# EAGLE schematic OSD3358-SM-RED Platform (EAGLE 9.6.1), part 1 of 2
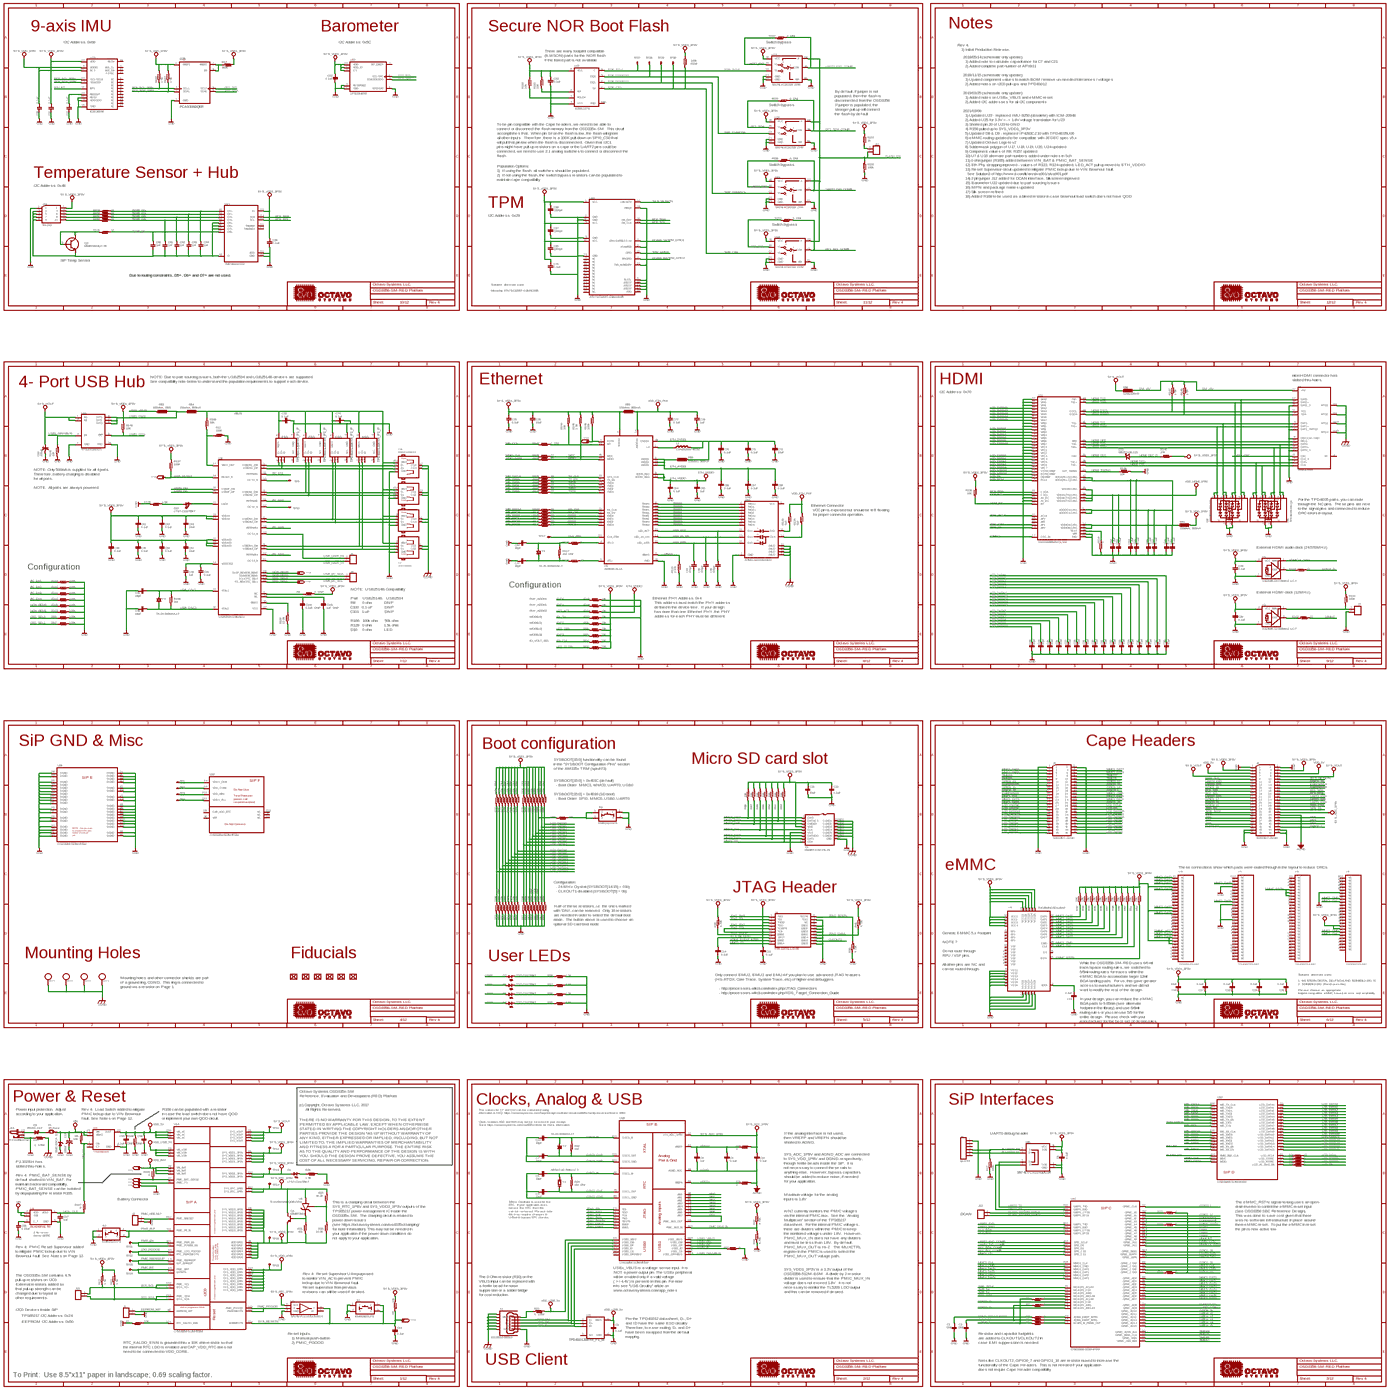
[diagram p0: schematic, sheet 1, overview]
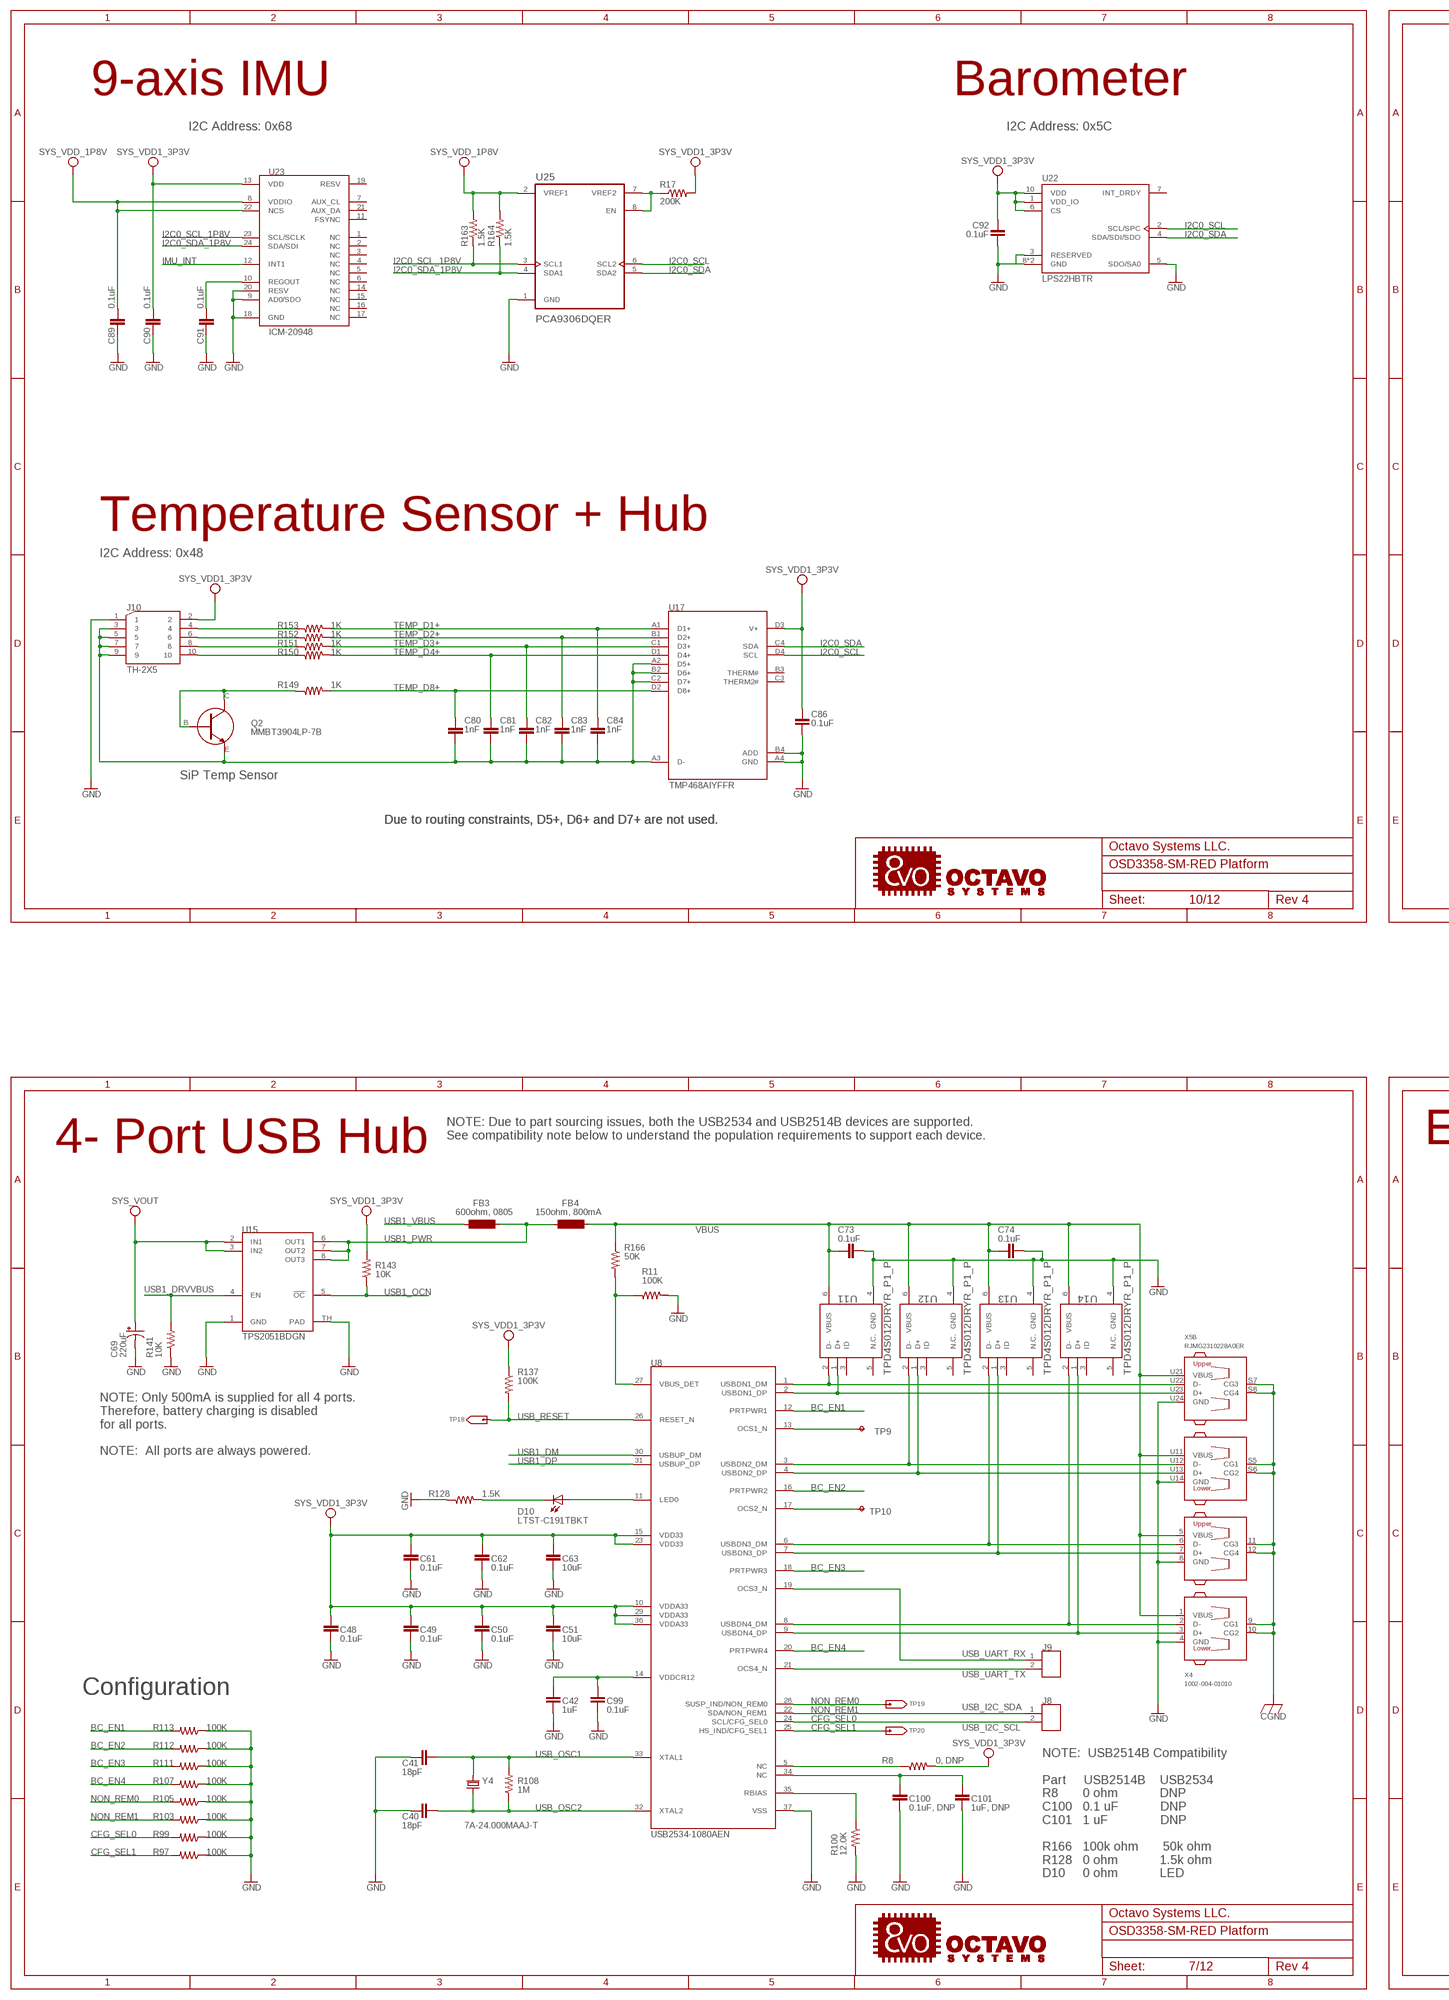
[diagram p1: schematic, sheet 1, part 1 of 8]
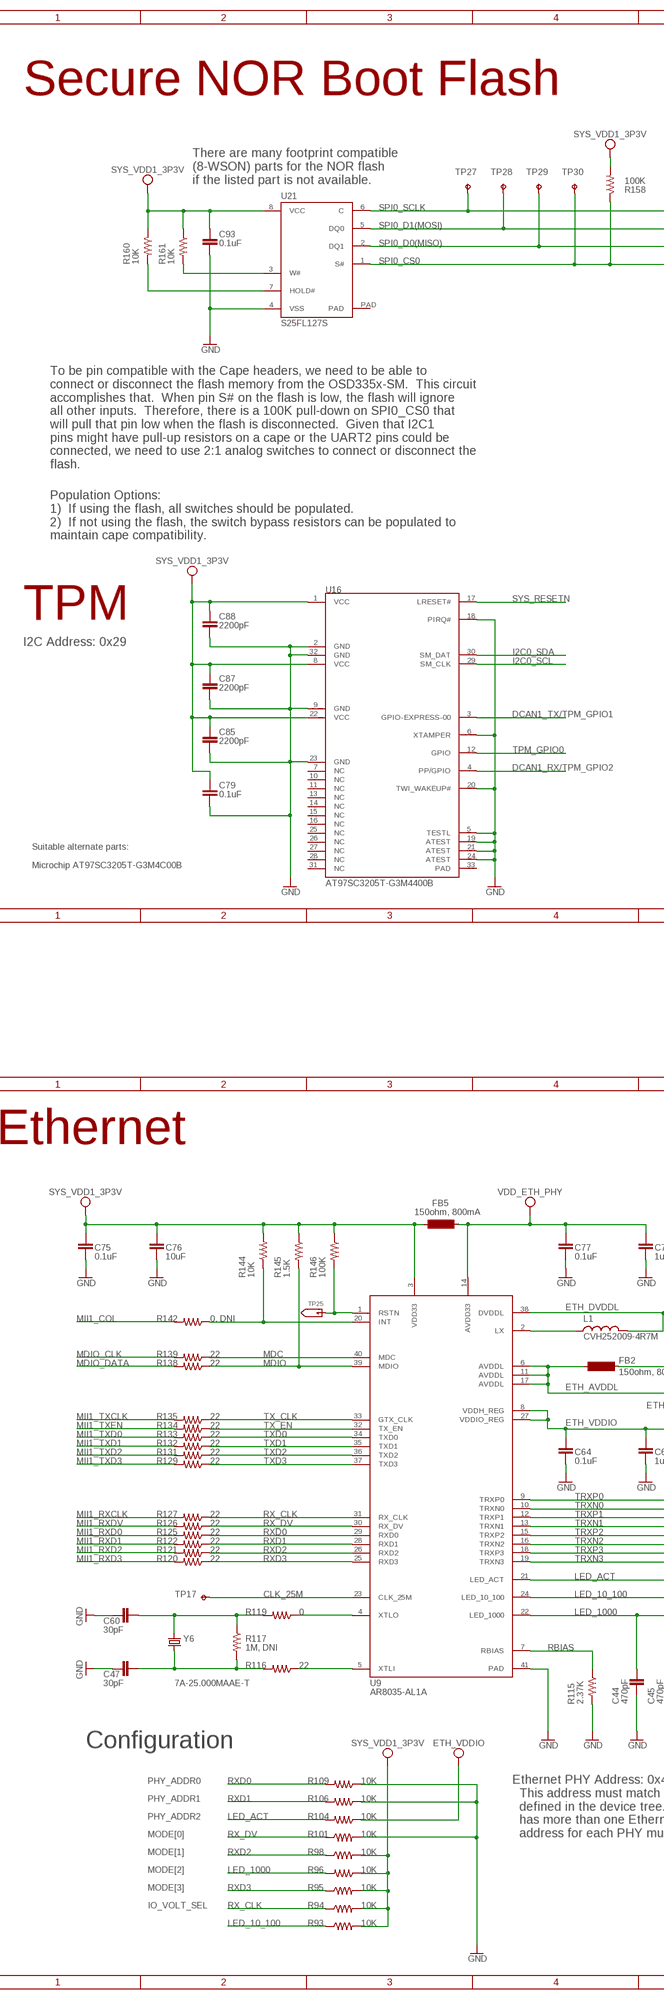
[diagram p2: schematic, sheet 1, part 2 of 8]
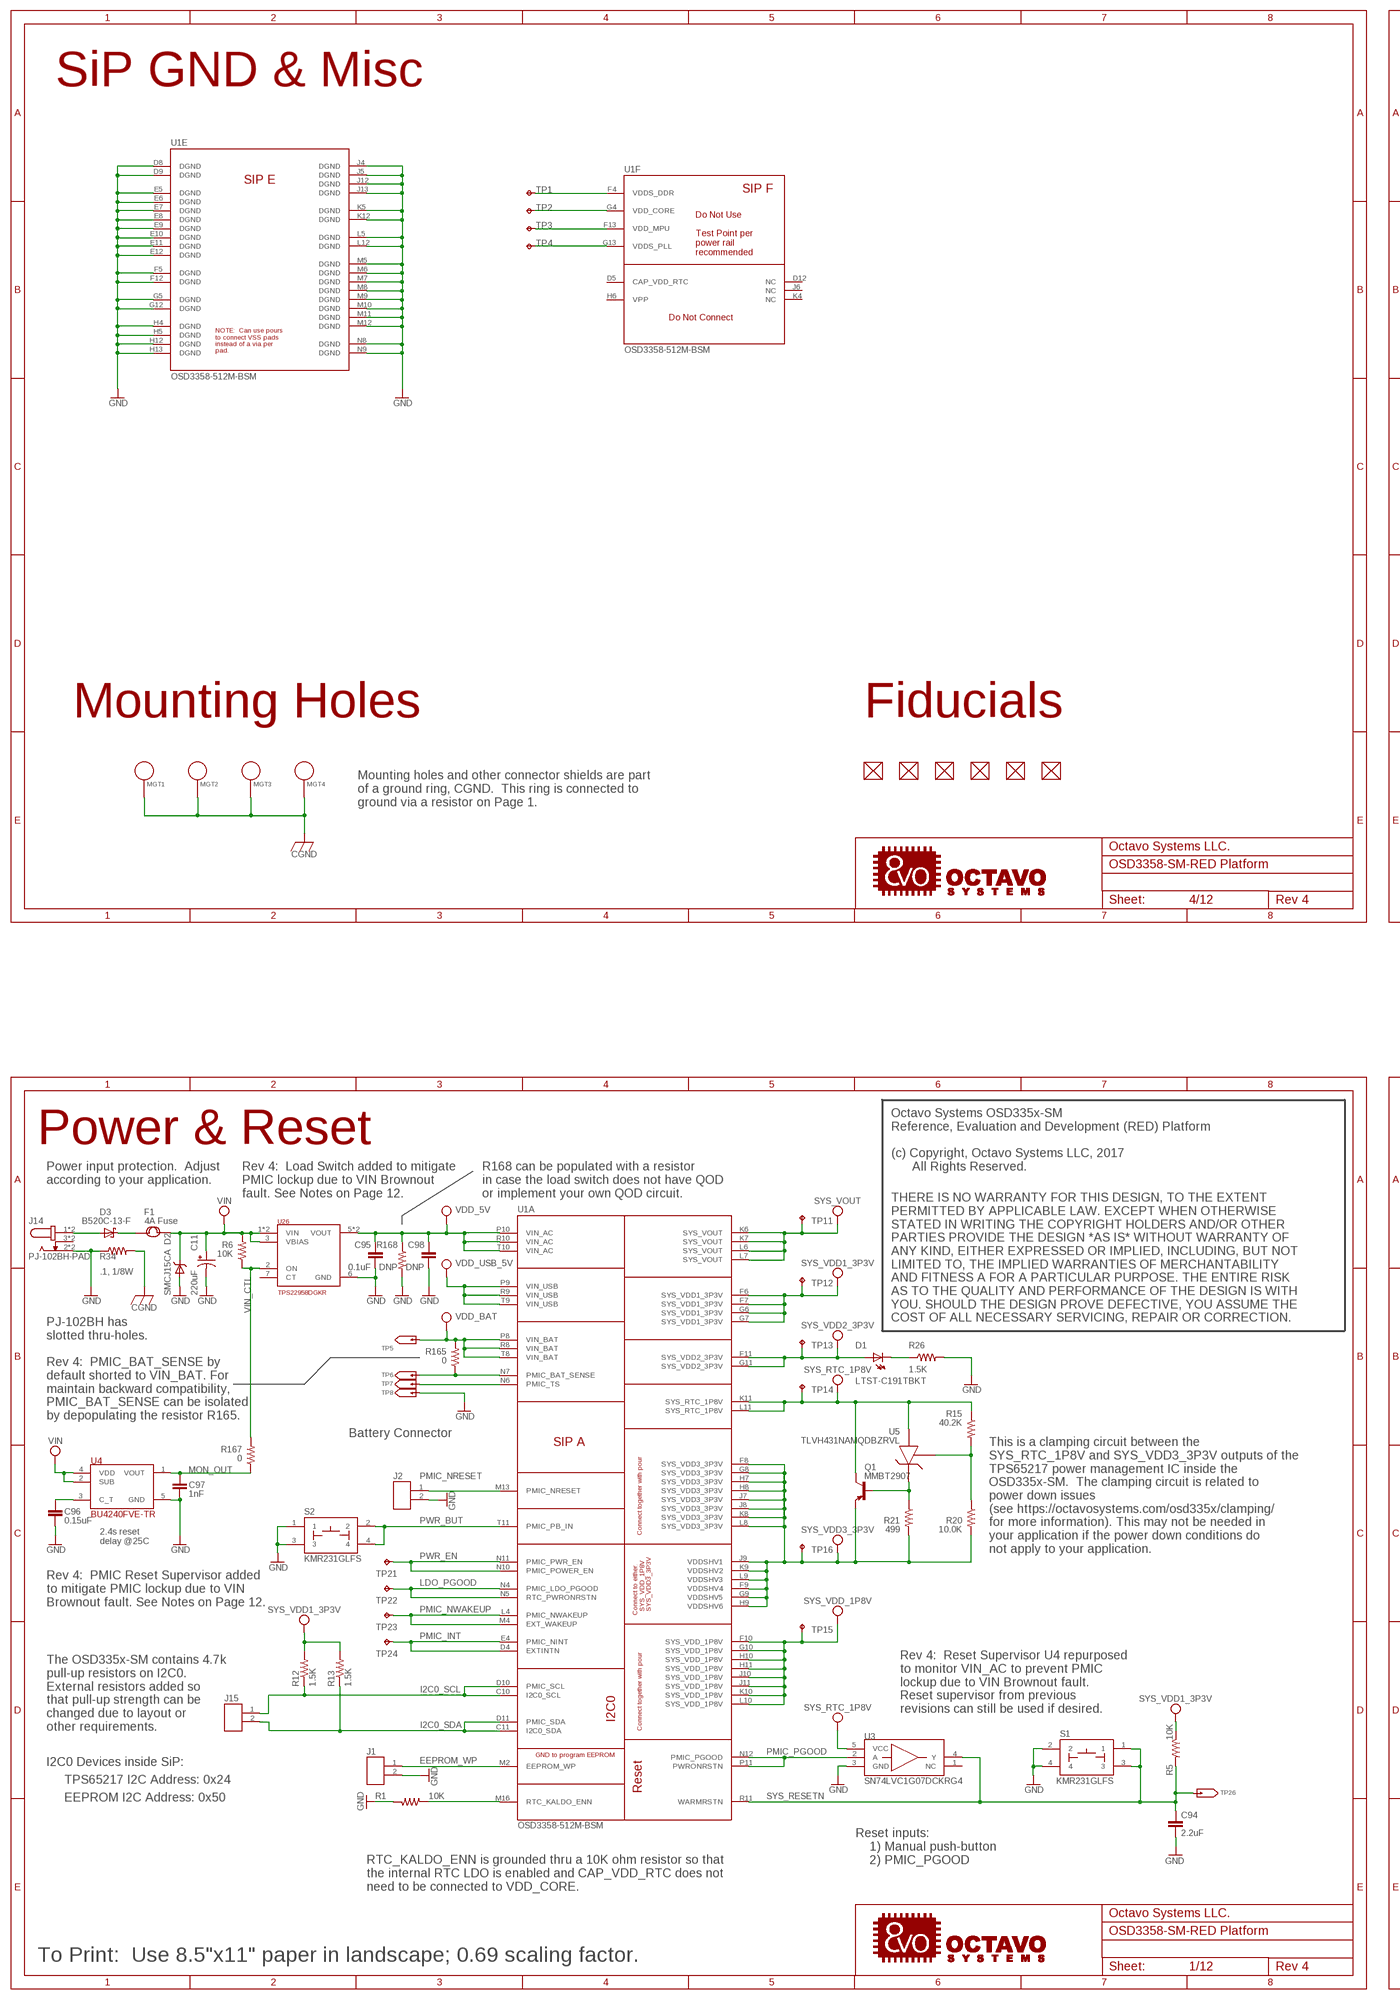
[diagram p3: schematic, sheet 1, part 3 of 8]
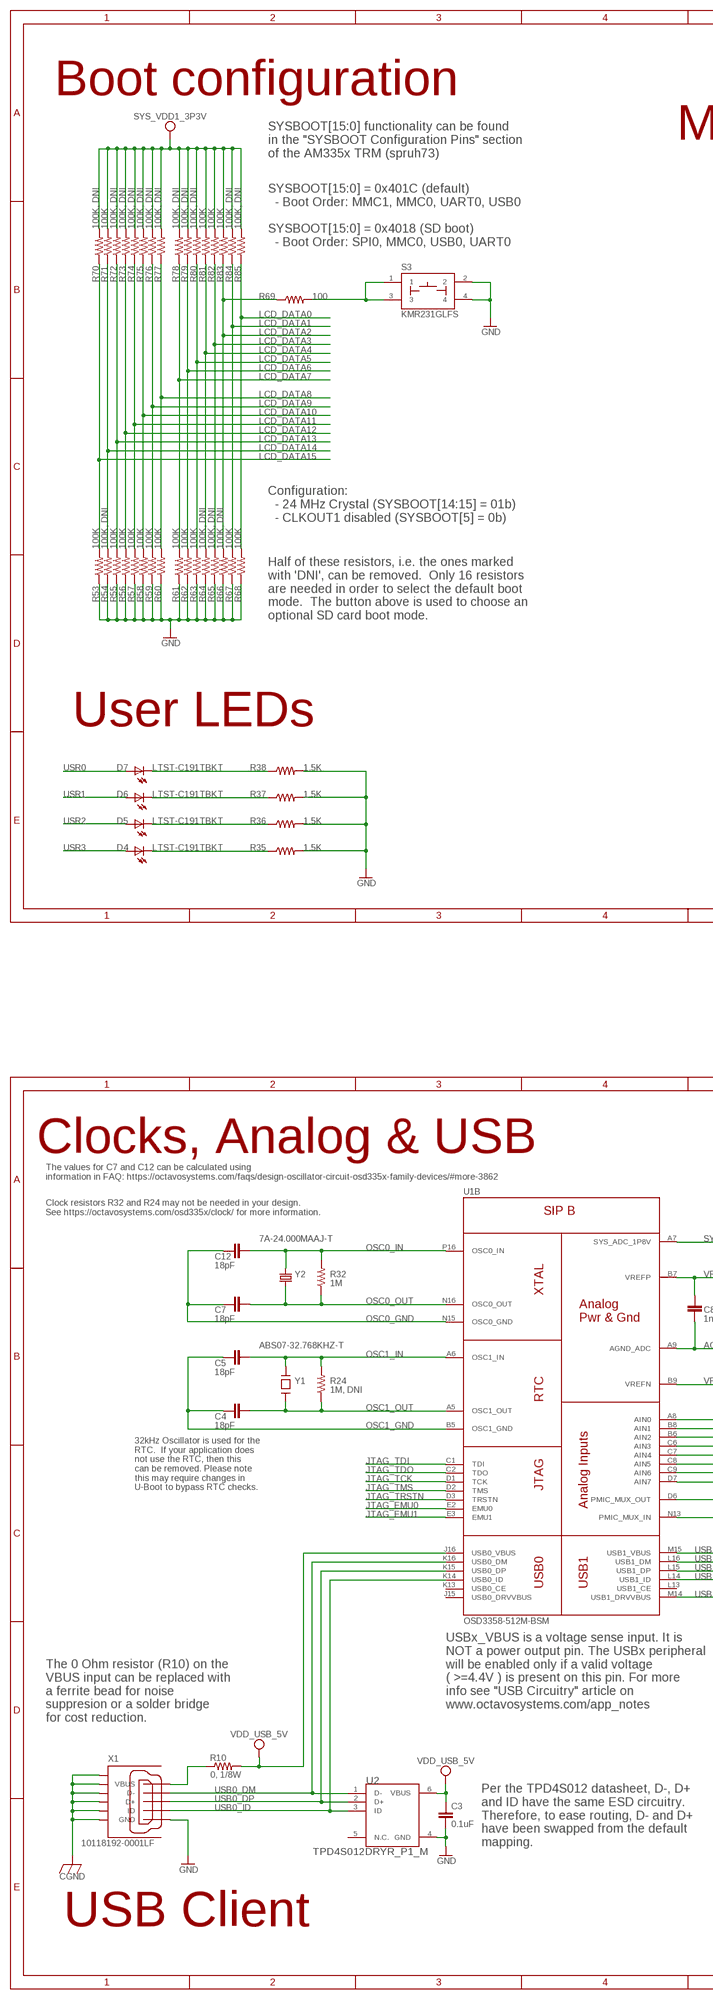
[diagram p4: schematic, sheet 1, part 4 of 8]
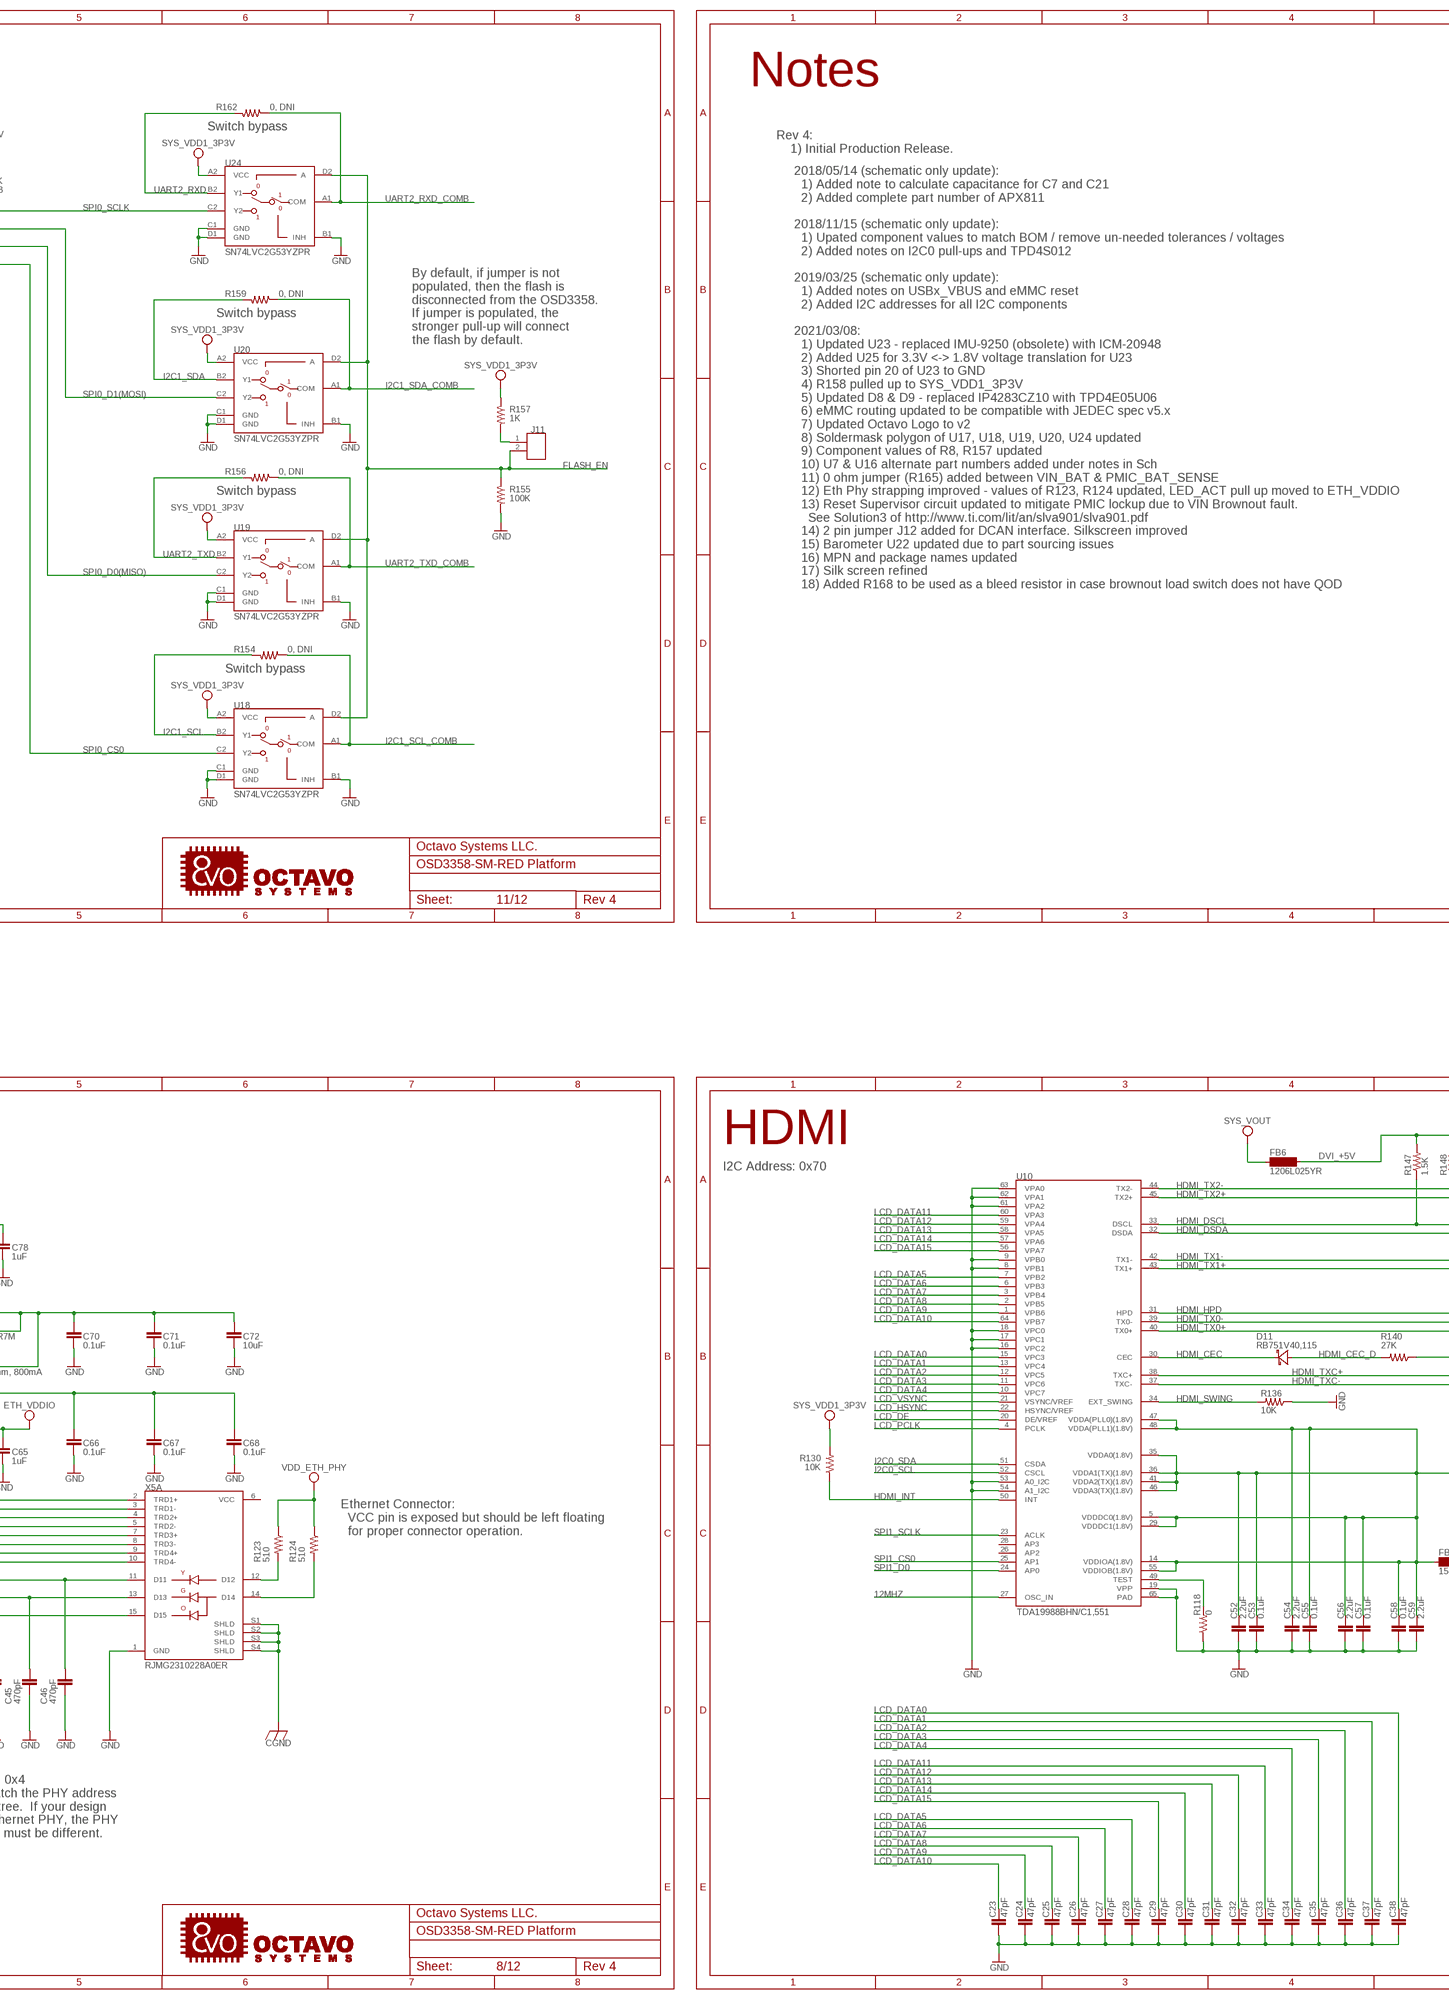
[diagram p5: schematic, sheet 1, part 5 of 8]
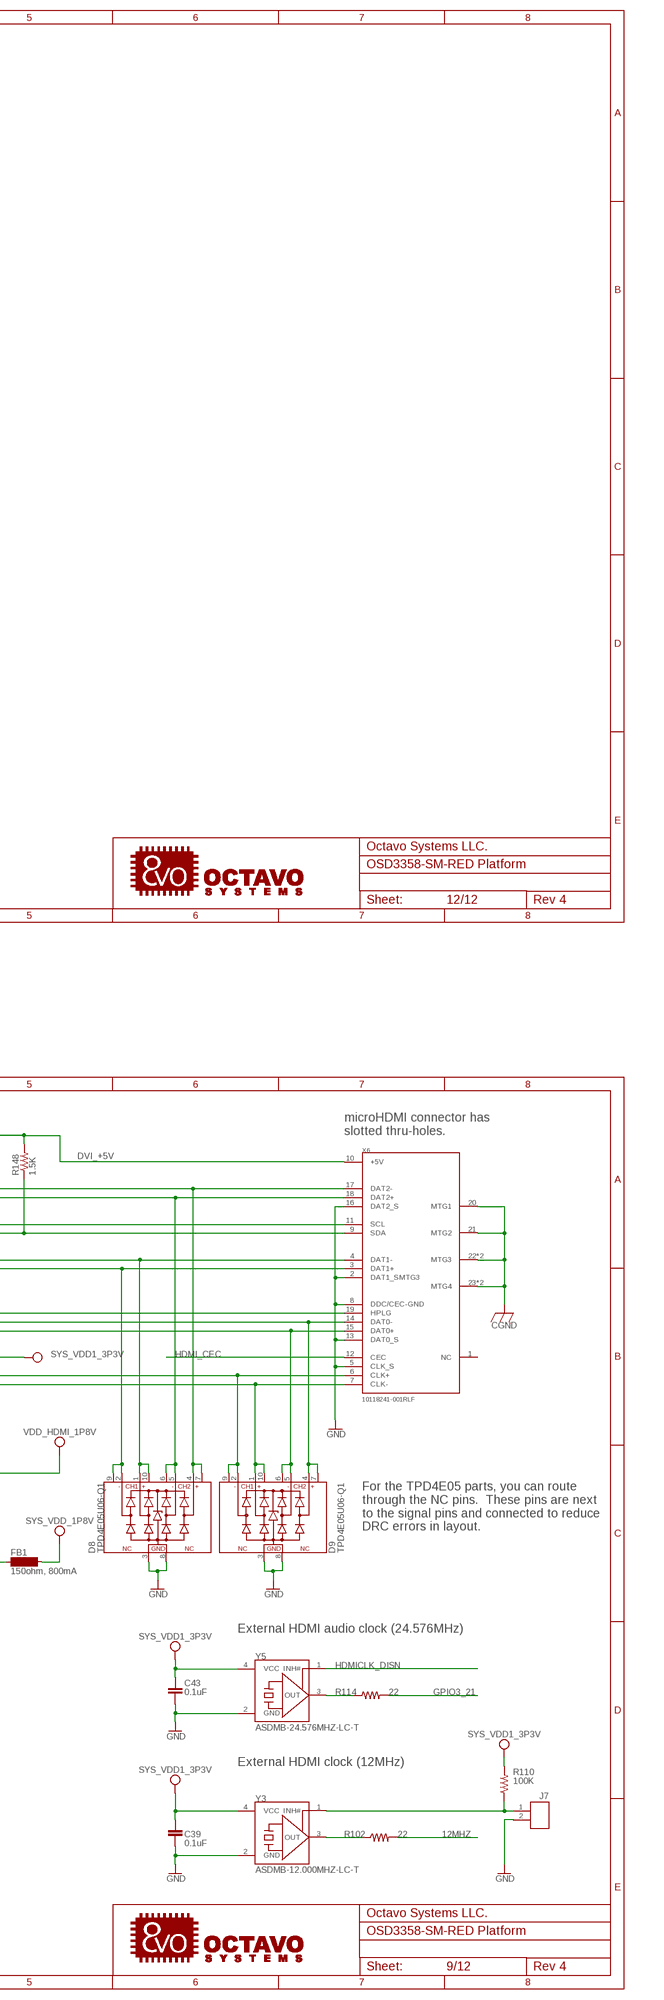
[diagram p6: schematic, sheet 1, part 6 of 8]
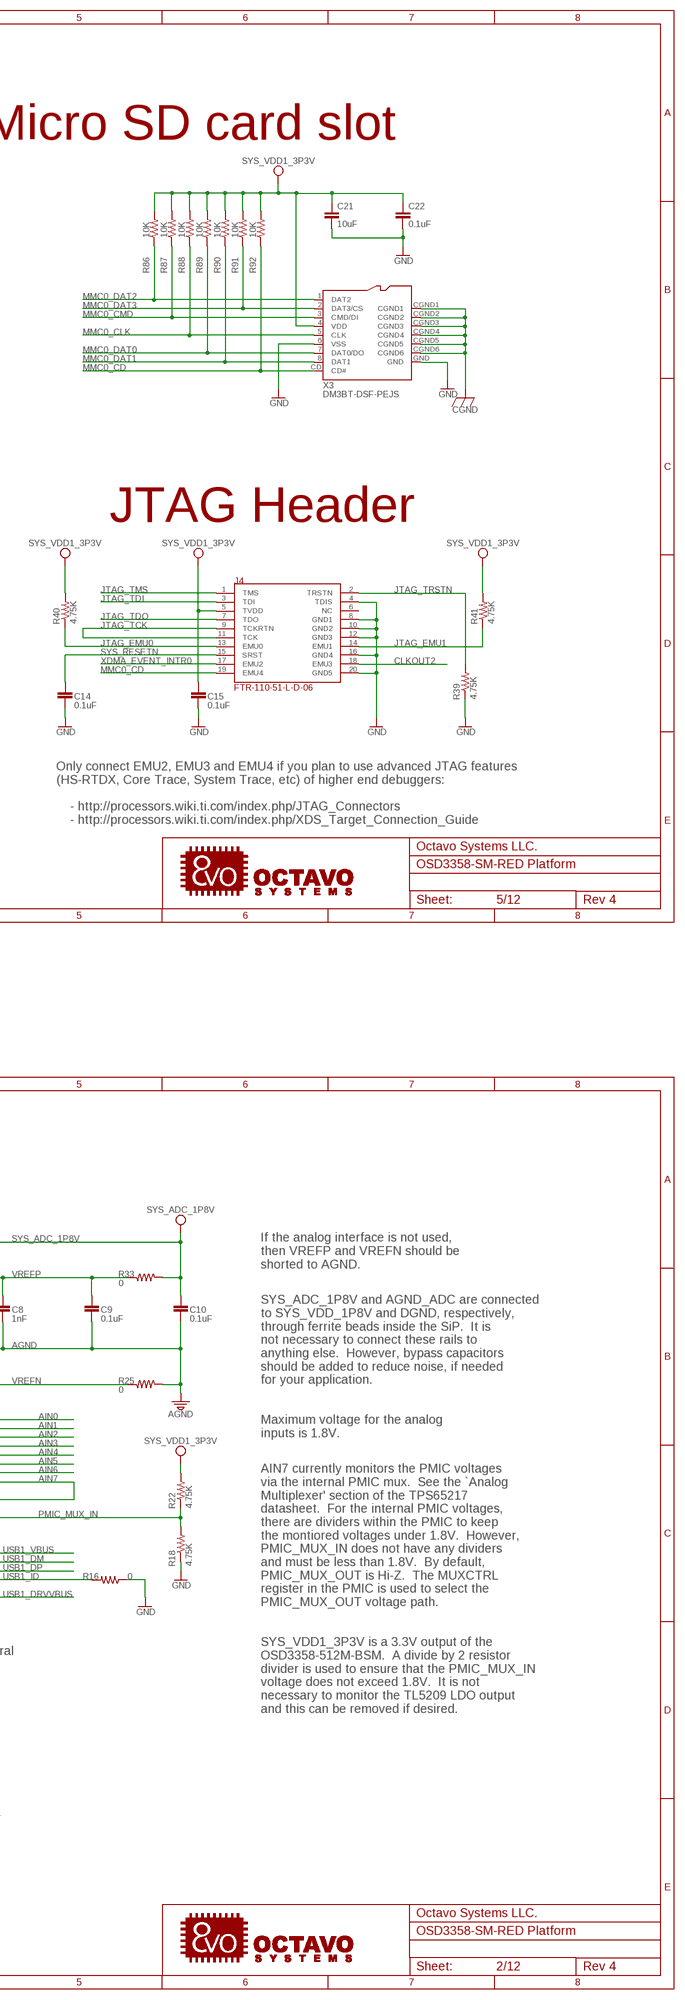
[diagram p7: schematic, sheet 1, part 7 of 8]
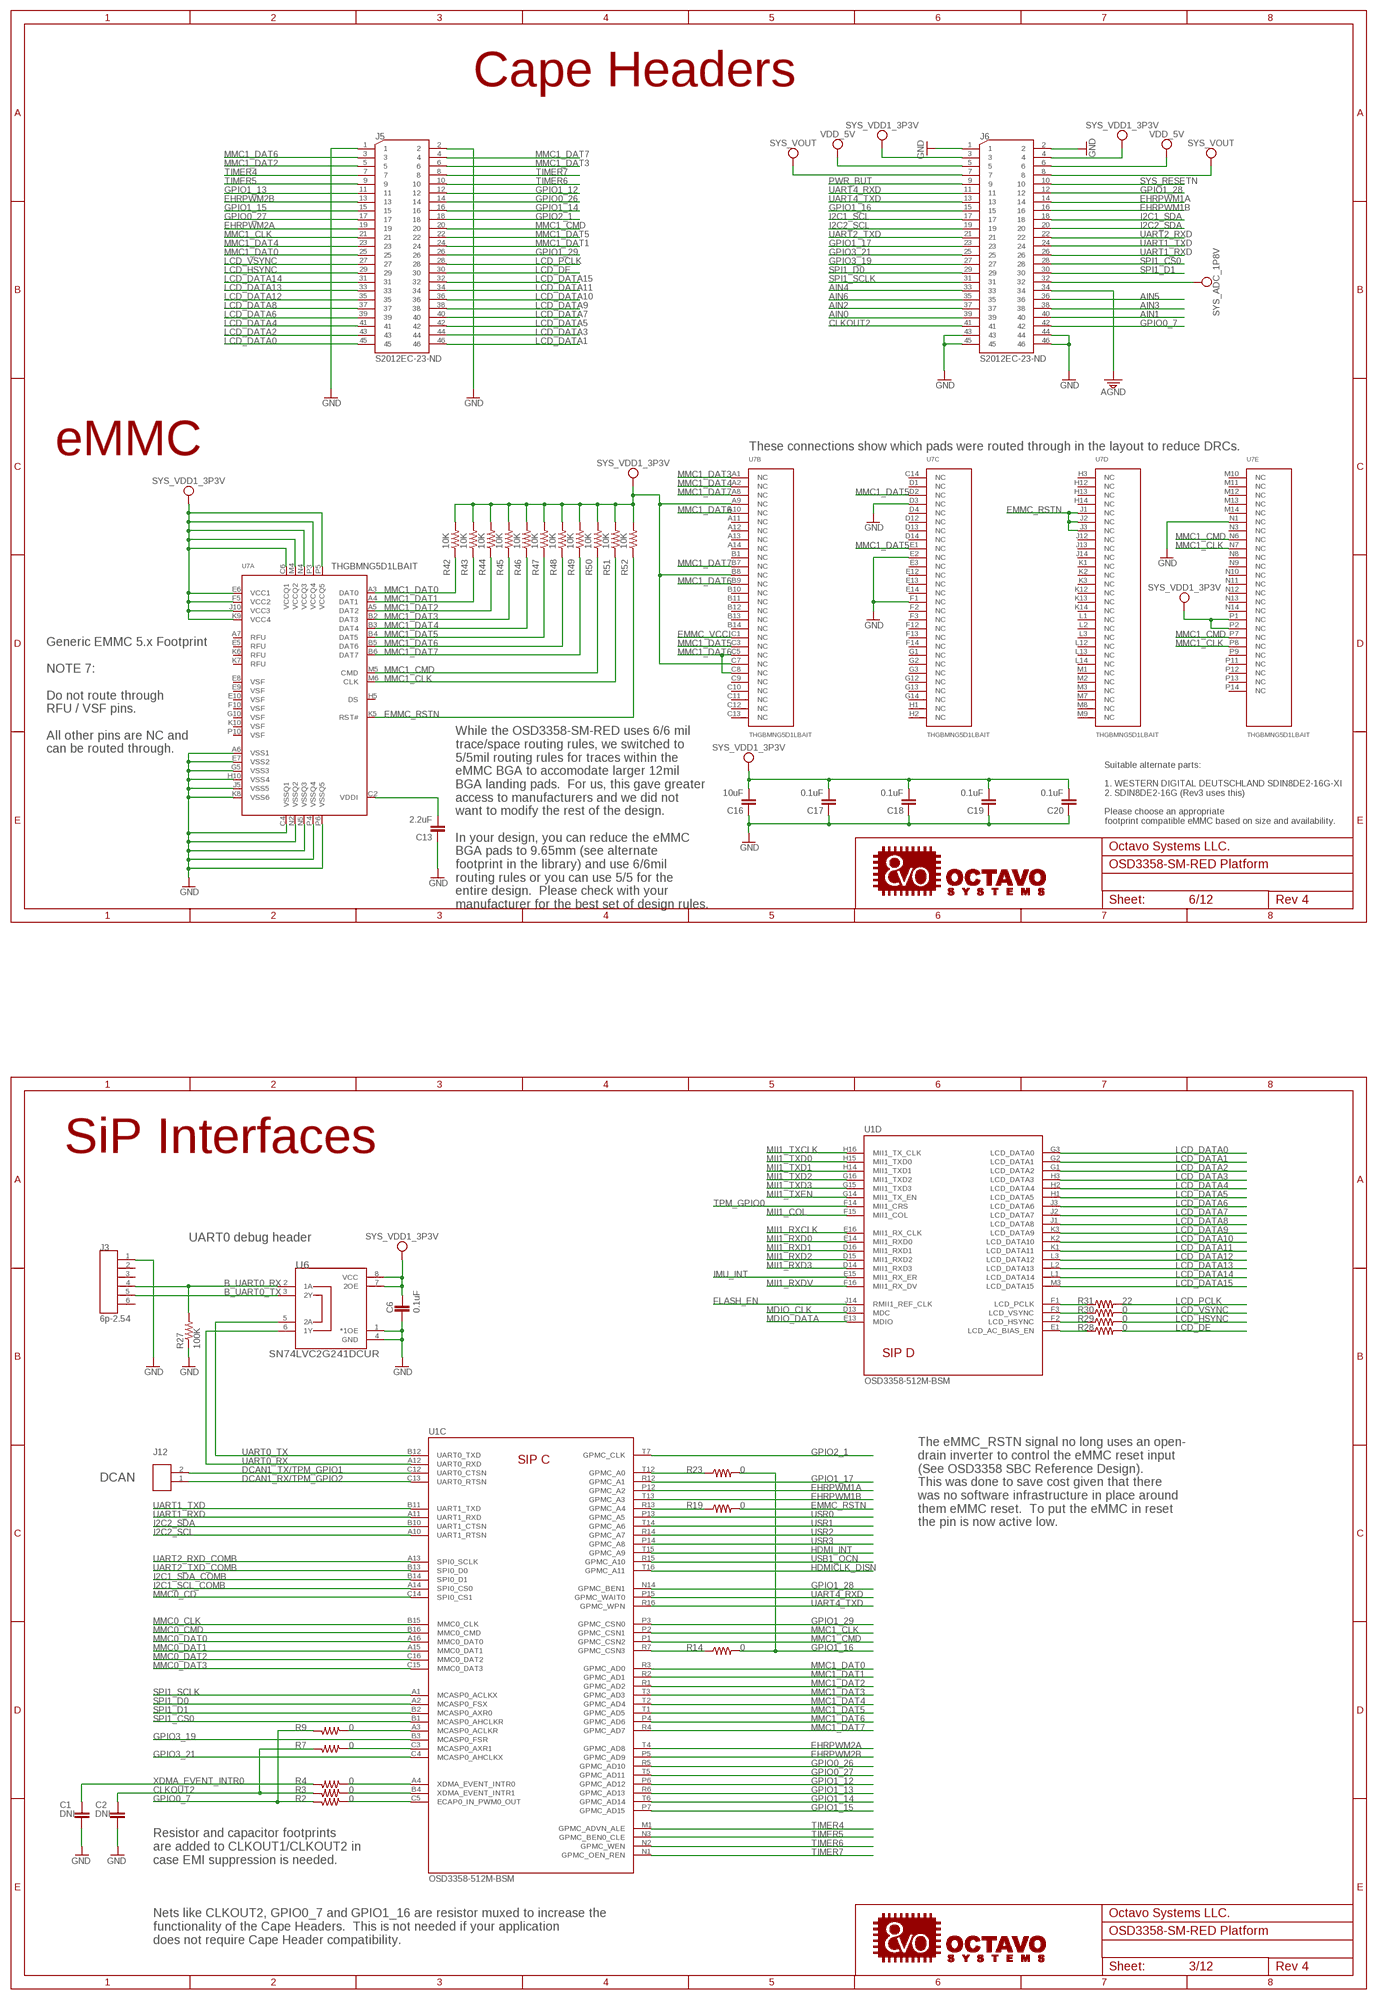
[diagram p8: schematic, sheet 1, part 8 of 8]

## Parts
C1  DNI  CC0603  [C0603]
C2  DNI  CC0603  [C0603]
C3  0.1uF  CC0402  [C0402]
C4  18pF  CC0402  [C0402]
C5  18pF  CC0402  [C0402]
C6  0.1uF  CC0402  [C0402]
C7  18pF  CC0402  [C0402]
C8  1nF  CC0402  [C0402]
C9  0.1uF  CC0402  [C0402]
C10  0.1uF  CC0402  [C0402]
C11  220uF  CPOL-USB/3528-21R  [B/3528-21R]
C12  18pF  CC0402  [C0402]
C13  2.2uF  CC0402  [C0402]
C14  0.1uF  CC0402  [C0402]
C15  0.1uF  CC0402  [C0402]
C16  10uF  CC0805  [C0805]
C17  0.1uF  CC0402  [C0402]
C18  0.1uF  CC0402  [C0402]
C19  0.1uF  CC0402  [C0402]
C20  0.1uF  CC0402  [C0402]
C21  10uF  CC0805  [C0805]
C22  0.1uF  CC0402  [C0402]
C23  47pF  CC0402  [C0402]
C24  47pF  CC0402  [C0402]
C25  47pF  CC0402  [C0402]
C26  47pF  CC0402  [C0402]
C27  47pF  CC0402  [C0402]
C28  47pF  CC0402  [C0402]
C29  47pF  CC0402  [C0402]
C30  47pF  CC0402  [C0402]
C31  47pF  CC0402  [C0402]
C32  47pF  CC0402  [C0402]
C33  47pF  CC0402  [C0402]
C34  47pF  CC0402  [C0402]
C35  47pF  CC0402  [C0402]
C36  47pF  CC0402  [C0402]
C37  47pF  CC0402  [C0402]
C38  47pF  CC0402  [C0402]
C39  0.1uF  CC0402  [C0402]
C40  18pF  CC0402  [C0402]
C41  18pF  CC0402  [C0402]
C42  1uF  CC0402  [C0402]
C43  0.1uF  CC0402  [C0402]
C44  470pF  CC0402  [C0402]
C45  470pF  CC0402  [C0402]
C46  470pF  CC0402  [C0402]
C47  30pF  CC0402  [C0402]
C48  0.1uF  CC0402  [C0402]
C49  0.1uF  CC0402  [C0402]
C50  0.1uF  CC0402  [C0402]
C51  10uF  CC0805  [C0805]
C52  2.2uF  CC0402  [C0402]
C53  0.1uF  CC0402  [C0402]
C54  2.2uF  CC0402  [C0402]
C55  0.1uF  CC0402  [C0402]
C56  2.2uF  CC0402  [C0402]
C57  0.1uF  CC0402  [C0402]
C58  0.1uF  CC0402  [C0402]
C59  2.2uF  CC0402  [C0402]
C60  30pF  CC0402  [C0402]
C61  0.1uF  CC0402  [C0402]
C62  0.1uF  CC0402  [C0402]
C63  10uF  CC0805  [C0805]
C64  0.1uF  CC0402  [C0402]
C65  1uF  CC0402  [C0402]
C66  0.1uF  CC0402  [C0402]
C67  0.1uF  CC0402  [C0402]
C68  0.1uF  CC0402  [C0402]
C69  220uF  CPOL-USB/3528-21R  [B/3528-21R]
C70  0.1uF  CC0402  [C0402]
C71  0.1uF  CC0402  [C0402]
C72  10uF  CC0805  [C0805]
C73  0.1uF  CC0402  [C0402]
C74  0.1uF  CC0402  [C0402]
C75  0.1uF  CC0402  [C0402]
C76  10uF  CC0805  [C0805]
C77  0.1uF  CC0402  [C0402]
C78  1uF  CC0402  [C0402]
C79  0.1uF  CC0402  [C0402]
C80  1nF  CC0402  [C0402]
C81  1nF  CC0402  [C0402]
C82  1nF  CC0402  [C0402]
C83  1nF  CC0402  [C0402]
C84  1nF  CC0402  [C0402]
C85  2200pF  CC0402  [C0402]
C86  0.1uF  CC0402  [C0402]
C87  2200pF  CC0402  [C0402]
C88  2200pF  CC0402  [C0402]
C89  0.1uF  CC0402  [C0402]
C90  0.1uF  CC0402  [C0402]
C91  0.1uF  CC0402  [C0402]
C92  0.1uF  CC0402  [C0402]
C93  0.1uF  CC0402  [C0402]
C94  2.2uF  CC0402  [C0402]
C95  0.1uF  CC0402  [C0402]
C96  0.15uF  CC0402  [C0402]
C97  1nF  CC0402  [C0402]
C98  DNP  CC0805  [C0805]
C99  0.1uF  CC0402  [C0402]
C100  0.1uF, DNP  CC0402  [C0402]
C101  1uF, DNP  CC0402  [C0402]
D1  LTST-C191TBKT  [0603]
D2  SMCJ15CA  [SMC]
D3  B520C-13-F  [SMC]
D4  LTST-C191TBKT  [0603]
D5  LTST-C191TBKT  [0603]
D6  LTST-C191TBKT  [0603]
D7  LTST-C191TBKT  [0603]
D8  TPD4E05U06-Q1  [10-USON(2.5X1)]
D9  TPD4E05U06-Q1  [10-USON(2.5X1)]
D10  LTST-C191TBKT  [0603]
D11  RB751V40,115  RB751V40-115SOD323-(REFLOW)  [SOD323(NXP)REFLOW]
F1  4A Fuse  FUSE'1206-WIDE'  [F1206W]
FB1  150ohm, 800mA  BLM21AG151SN1DFB_0805  [C0805]
FB2  150ohm, 800mA  BLM21AG151SN1DFB_0805  [C0805]
FB3  600ohm, 0805  MPZ2012S601AT000FB_0805  [C0805]
FB4  150ohm, 800mA  BLM21AG151SN1DFB_0805  [C0805]
FB5  150ohm, 800mA  BLM21AG151SN1DFB_0805  [C0805]
FB6  1206L025YR  MPZ2012S601AT000FB_1206  [SM-1206]
FUD1  FIDUCIAL  [FIDUCIAL_40MIL]
FUD2  FIDUCIAL  [FIDUCIAL_40MIL]
FUD3  FIDUCIAL  [FIDUCIAL_40MIL]
FUD4  FIDUCIAL  [FIDUCIAL_40MIL]
FUD5  FIDUCIAL  [FIDUCIAL_40MIL]
FUD6  FIDUCIAL  [FIDUCIAL_40MIL]
J1  826646-2  [H2-2.54]
J2  826646-2  [H2-2.54]
J3  6p-2.54  826646-6  [H6-2.54]
J4  FTR-110-51-L-D-06  [2ROWS_10PINS_1.27MM_PITCH_ROW_2.54MM_PITCH_PIN6_KEYED]
J5  S2012EC-23-ND  TH-2X23  [H2X23-2.54]
J6  S2012EC-23-ND  TH-2X23  [H2X23-2.54]
J7  826646-2  [H2-2.54]
J8  826646-2  [H2-2.54]
J9  826646-2  [H2-2.54]
J10  TH-2X5  [H2X5-2.54]
J11  826646-2  [H2-2.54]
J12  826646-2  [H2-2.54]
J14  PJ-102BH-PAD  [CUI_PJ-102BH-DIM-SMT-PAD]
J15  826646-2  [H2-2.54]
L1  CVH252009-4R7M  [CVH252009]
MGT1  MOUNTING_HOLE  [MOUNTING_HOLE]
MGT2  MOUNTING_HOLE  [MOUNTING_HOLE]
MGT3  MOUNTING_HOLE  [MOUNTING_HOLE]
MGT4  MOUNTING_HOLE  [MOUNTING_HOLE]
Q1  MMBT2907  [SOT23-BEC]
Q2  MMBT3904LP-7B  [X1-DFN1006-3]
R1  10K  R-US_R0402  [R0402]
R2  0  R-US_R0402  [R0402]
R3  0  R-US_R0402  [R0402]
R4  0  R-US_R0402  [R0402]
R5  10K  R-US_R0402  [R0402]
R6  10K  R-US_R0402  [R0402]
R7  0  R-US_R0402  [R0402]
R8  0, DNP  R-US_R0402  [R0402]
R9  0  R-US_R0402  [R0402]
R10  0, 1/8W  R-US_R0805  [R0805]
R11  100K  R-US_R0402  [R0402]
R12  1.5K  R-US_R0402  [R0402]
R13  1.5K  R-US_R0402  [R0402]
R14  0  R-US_R0402  [R0402]
R15  40.2K  R-US_R0402  [R0402]
R16  0  R-US_R0402  [R0402]
R17  200K  R-US_R0402  [R0402]
R18  4.75K  R-US_R0402  [R0402]
R19  0  R-US_R0402  [R0402]
R20  10.0K  R-US_R0402  [R0402]
R21  499  R-US_R0402  [R0402]
R22  4.75K  R-US_R0402  [R0402]
R23  0  R-US_R0402  [R0402]
R24  1M, DNI  R-US_R0402  [R0402]
R25  0  R-US_R0402  [R0402]
R26  1.5K  R-US_R0402  [R0402]
R27  100K  R-US_R0402  [R0402]
R28  0  R-US_R0402  [R0402]
R29  0  R-US_R0402  [R0402]
R30  0  R-US_R0402  [R0402]
R31  22  R-US_R0402  [R0402]
R32  1M  R-US_R0402  [R0402]
R33  0  R-US_R0402  [R0402]
R34  .1, 1/8W  R-US_R0805  [R0805]
R35  1.5K  R-US_R0402  [R0402]
R36  1.5K  R-US_R0402  [R0402]
R37  1.5K  R-US_R0402  [R0402]
R38  1.5K  R-US_R0402  [R0402]
R39  4.75K  R-US_R0402  [R0402]
R40  4.75K  R-US_R0402  [R0402]
R41  4.75K  R-US_R0402  [R0402]
R42  10K  R-US_R0402  [R0402]
R43  10K  R-US_R0402  [R0402]
R44  10K  R-US_R0402  [R0402]
R45  10K  R-US_R0402  [R0402]
R46  10K  R-US_R0402  [R0402]
R47  10K  R-US_R0402  [R0402]
R48  10K  R-US_R0402  [R0402]
R49  10K  R-US_R0402  [R0402]
R50  10K  R-US_R0402  [R0402]
R51  10K  R-US_R0402  [R0402]
R52  10K  R-US_R0402  [R0402]
R53  100K  R-US_R0402  [R0402]
R54  100K, DNI  R-US_R0402  [R0402]
R55  100K  R-US_R0402  [R0402]
R56  100K  R-US_R0402  [R0402]
R57  100K  R-US_R0402  [R0402]
R58  100K  R-US_R0402  [R0402]
R59  100K  R-US_R0402  [R0402]
R60  100K  R-US_R0402  [R0402]
R61  100K  R-US_R0402  [R0402]
R62  100K  R-US_R0402  [R0402]
R63  100K  R-US_R0402  [R0402]
R64  100K, DNI  R-US_R0402  [R0402]
R65  100K, DNI  R-US_R0402  [R0402]
R66  100K, DNI  R-US_R0402  [R0402]
R67  100K  R-US_R0402  [R0402]
R68  100K  R-US_R0402  [R0402]
R69  100  R-US_R0402  [R0402]
R70  100K, DNI  R-US_R0402  [R0402]
R71  100K  R-US_R0402  [R0402]
R72  100K, DNI  R-US_R0402  [R0402]
R73  100K, DNI  R-US_R0402  [R0402]
R74  100K, DNI  R-US_R0402  [R0402]
R75  100K, DNI  R-US_R0402  [R0402]
R76  100K, DNI  R-US_R0402  [R0402]
R77  100K, DNI  R-US_R0402  [R0402]
R78  100K, DNI  R-US_R0402  [R0402]
R79  100K, DNI  R-US_R0402  [R0402]
R80  100K, DNI  R-US_R0402  [R0402]
R81  100K  R-US_R0402  [R0402]
R82  100K  R-US_R0402  [R0402]
R83  100K  R-US_R0402  [R0402]
R84  100K, DNI  R-US_R0402  [R0402]
R85  100K, DNI  R-US_R0402  [R0402]
R86  10K  R-US_R0402  [R0402]
R87  10K  R-US_R0402  [R0402]
R88  10K  R-US_R0402  [R0402]
R89  10K  R-US_R0402  [R0402]
R90  10K  R-US_R0402  [R0402]
R91  10K  R-US_R0402  [R0402]
R92  10K  R-US_R0402  [R0402]
R93  10K  R-US_R0402  [R0402]
R94  10K  R-US_R0402  [R0402]
R95  10K  R-US_R0402  [R0402]
R96  10K  R-US_R0402  [R0402]
R97  100K  R-US_R0402  [R0402]
R98  10K  R-US_R0402  [R0402]
R99  100K  R-US_R0402  [R0402]
R100  12.0K  R-US_R0402  [R0402]
R101  10K  R-US_R0402  [R0402]
R102  22  R-US_R0402  [R0402]
R103  100K  R-US_R0402  [R0402]
R104  10K  R-US_R0402  [R0402]
R105  100K  R-US_R0402  [R0402]
R106  10K  R-US_R0402  [R0402]
R107  100K  R-US_R0402  [R0402]
R108  1M  R-US_R0402  [R0402]
R109  10K  R-US_R0402  [R0402]
R110  100K  R-US_R0402  [R0402]
R111  100K  R-US_R0402  [R0402]
R112  100K  R-US_R0402  [R0402]
R113  100K  R-US_R0402  [R0402]
R114  22  R-US_R0402  [R0402]
R115  2.37K  R-US_R0402  [R0402]
R116  22  R-US_R0402  [R0402]
R117  1M, DNI  R-US_R0402  [R0402]
R118  0  R-US_R0402  [R0402]
R119  0  R-US_R0402  [R0402]
R120  22  R-US_R0402  [R0402]
R121  22  R-US_R0402  [R0402]
R122  22  R-US_R0402  [R0402]
R123  510  R-US_R0402  [R0402]
R124  510  R-US_R0402  [R0402]
R125  22  R-US_R0402  [R0402]
R126  22  R-US_R0402  [R0402]
R127  22  R-US_R0402  [R0402]
R128  1.5K  R-US_R0402  [R0402]
R129  22  R-US_R0402  [R0402]
R130  10K  R-US_R0402  [R0402]
R131  22  R-US_R0402  [R0402]
R132  22  R-US_R0402  [R0402]
R133  22  R-US_R0402  [R0402]
R134  22  R-US_R0402  [R0402]
R135  22  R-US_R0402  [R0402]
R136  10K  R-US_R0402  [R0402]
R137  100K  R-US_R0402  [R0402]
R138  22  R-US_R0402  [R0402]
R139  22  R-US_R0402  [R0402]
R140  27K  R-US_R0402  [R0402]
R141  10K  R-US_R0402  [R0402]
R142  0, DNI  R-US_R0402  [R0402]
R143  10K  R-US_R0402  [R0402]
R144  10K  R-US_R0402  [R0402]
R145  1.5K  R-US_R0402  [R0402]
R146  100K  R-US_R0402  [R0402]
R147  1.5K  R-US_R0402  [R0402]
R148  1.5K  R-US_R0402  [R0402]
R149  1K  R-US_R0402  [R0402]
R150  1K  R-US_R0402  [R0402]
R151  1K  R-US_R0402  [R0402]
R152  1K  R-US_R0402  [R0402]
R153  1K  R-US_R0402  [R0402]
R154  0, DNI  R-US_R0402  [R0402]
R155  100K  R-US_R0402  [R0402]
R156  0, DNI  R-US_R0402  [R0402]
R157  1K  R-US_R0402  [R0402]
R158  100K  R-US_R0402  [R0402]
R159  0, DNI  R-US_R0402  [R0402]
R160  10K  R-US_R0402  [R0402]
R161  10K  R-US_R0402  [R0402]
R162  0, DNI  R-US_R0402  [R0402]
R163  1.5K  R-US_R0402  [R0402]
R164  1.5K  R-US_R0402  [R0402]
R165  0  R-US_R0402  [R0402]
R166  50K  R-US_R0402  [R0402]
R167  0  R-US_R0402  [R0402]
R168  DNP  R-US_R0805  [R0805]
S1  KMR231GLFS  [SW4SMD_63X161LS]
S2  KMR231GLFS  [SW4SMD_63X161LS]
S3  KMR231GLFS  [SW4SMD_63X161LS]
TP1  TPB0,65  [TP_B0,65]
TP2  TPB0,65  [TP_B0,65]
TP3  TPB0,65  [TP_B0,65]
TP4  TPB0,65  [TP_B0,65]
TP5  TESTPAD/W_HOLE_1X1  [TESTPAD/W_HOLE_1X1]
TP6  TESTPAD/W_HOLE_1X1  [TESTPAD/W_HOLE_1X1]
TP7  TESTPAD/W_HOLE_1X1  [TESTPAD/W_HOLE_1X1]
TP8  TESTPAD/W_HOLE_1X1  [TESTPAD/W_HOLE_1X1]
TP9  TPB0,65  [TP_B0,65]
TP10  TPB0,65  [TP_B0,65]
TP11  TPB0,65  [TP_B0,65]
TP12  TPB0,65  [TP_B0,65]
TP13  TPB0,65  [TP_B0,65]
TP14  TPB0,65  [TP_B0,65]
TP15  TPB0,65  [TP_B0,65]
TP16  TPB0,65  [TP_B0,65]
TP17  TPB0,65  [TP_B0,65]
TP18  TESTPAD/W_HOLE_1X1  [TESTPAD/W_HOLE_1X1]
TP19  TESTPAD/W_HOLE_1X1  [TESTPAD/W_HOLE_1X1]
TP20  TESTPAD/W_HOLE_1X1  [TESTPAD/W_HOLE_1X1]
TP21  TPB0,65  [TP_B0,65]
TP22  TPB0,65  [TP_B0,65]
TP23  TPB0,65  [TP_B0,65]
TP24  TPB0,65  [TP_B0,65]
TP25  TESTPAD/W_HOLE_1X1  [TESTPAD/W_HOLE_1X1]
TP26  TESTPAD/W_HOLE_1X1  [TESTPAD/W_HOLE_1X1]
TP27  TPB0,65  [TP_B0,65]
TP28  TPB0,65  [TP_B0,65]
TP29  TPB0,65  [TP_B0,65]
TP30  TPB0,65  [TP_B0,65]
U1  OSD3358-512M-BSM  [OSD335X-BGA-256]
U2  TPD4S012DRYR_P1_M  [6-SON(1.45X1)]
U3  SN74LVC1G07DCKRG4  [SC-70-5]
U4  BU4240FVE-TR  [5-VSOF(1.6X1.6MM)]
U5  TLVH431NAMQDBZRVL  [SOT23-3]
U6  SN74LVC2G241DCUR  [8-VSSOP(2.3X2MM)]
U7  THGBMNG5D1LBAIT  [153-WFBGA(11X10)]
U8  USB2534-1080AEN  [6-SQFN(6X6)]
U9  AR8035-AL1A  [40-QFN(5X5MM)]
U10  TDA19988BHN/C1,551  [64-HVQFN(9X9)]
U11  TPD4S012DRYR_P1_P  [6-SON(1.45X1)]
U12  TPD4S012DRYR_P1_P  [6-SON(1.45X1)]
U13  TPD4S012DRYR_P1_P  [6-SON(1.45X1)]
U14  TPD4S012DRYR_P1_P  [6-SON(1.45X1)]
U15  TPS2051BDGN  [8-TSSOP(3.00MM_WIDTH)]
U16  AT97SC3205T-G3M4400B  [QFN32-0.4-4X4MM]
U17  TMP468AIYFFR  [16-DSBGA]
U18  SN74LVC2G53YZPR  [8-DSBGA(1.9X0.9)]
U19  SN74LVC2G53YZPR  [8-DSBGA(1.9X0.9)]
U20  SN74LVC2G53YZPR  [8-DSBGA(1.9X0.9)]
U21  S25FL127S  [8-WSON(5X6MM)]
U22  LPS22HBTR  [10-HLGA(2X2MM)]
U23  ICM-20948  [24-QFN(3X3)]
U24  SN74LVC2G53YZPR  [8-DSBGA(1.9X0.9)]
U25  PCA9306DQER  [8-X2SON(1.4X1.0)]
U26  TPS22958DGKR  [8-VSSOP(3X3MM)]
X1  10118192-0001LF  [MICRO_USB_2.0_RECEP_5POS_SMD_RIGHT_ANGLE]
X3  DM3BT-DSF-PEJS  [10(8+2)POS_MICRO_SD_SMD_RIGHT_ANGLE]
X4  1002-004-01010  [USB_HOST_HORIZONTAL_W/CHASSIS_GND_DUAL]
X5  RJMG2310228A0ER  [RJ45_10/100/1000_DUAL_USB_A_THRUHOLE_CONN]
X6  10118241-001RLF  [MICRO_HDMI_19POS_SMD&THRUHOLE_RIGHT_ANGLE]
Y1  ABS07-32.768KHZ-T  [2-SMD,NO_LEAD(3.2X1.5MM)]
Y2  7A-24.000MAAJ-T  [2-SMD,NO_LEAD(5X3.2MM)]
Y3  ASDMB-12.000MHZ-LC-T  [4-SMD,NO_LEAD(2.5X2MM)]
Y4  7A-24.000MAAJ-T  [2-SMD,NO_LEAD(5X3.2MM)]
Y5  ASDMB-24.576MHZ-LC-T  [4-SMD,NO_LEAD(2.5X2MM)]
Y6  7A-25.000MAAE-T  [2-SMD,NO_LEAD(5X3.2MM)]

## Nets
12MHZ: R102.2 U10.27(OSC_IN)
AGND: C8.2 C9.2 C10.2 J6.34 R25.2 U1.A9(B:AGND_ADC)
AIN0: J6.39 U1.A8(B:AIN0)
AIN1: J6.40 U1.B8(B:AIN1)
AIN2: J6.37 U1.B6(B:AIN2)
AIN3: J6.38 U1.C6(B:AIN3)
AIN4: J6.33 U1.C7(B:AIN4)
AIN5: J6.36 U1.C8(B:AIN5)
AIN6: J6.35 U1.C9(B:AIN6)
AIN7: U1.D6(B:PMIC_MUX_OUT) U1.D7(B:AIN7)
B_UART0_RX: J3.4 R27.2 U6.2(1A)
B_UART0_TX: J3.5 U6.3(2Y)
BAT_SENSE: R165.1 TP6.P$1(TP) U1.N7(A:PMIC_BAT_SENSE)
BC_EN1: R113.2 U8.12(PRTPWR1)
BC_EN2: R112.2 U8.16(PRTPWR2)
BC_EN3: R111.2 U8.18(PRTPWR3)
BC_EN4: R107.2 U8.20(PRTPWR4)
CFG_SEL0: J8.2 R99.2 U8.24(SCL/CFG_SEL0)
CFG_SEL1: R97.2 TP20.P$1(TP) U8.25(HS_IND/CFG_SEL1)
CGND: MGT1.P$1 MGT2.P$1 MGT3.P$1 MGT4.P$1 R34.2 X1.CGND1(SGND1) X1.CGND2(SGND2) X1.CGND3(SGND3) X1.CGND4(SGND4) X1.CGND5(SGND5) X1.CGND6(SGND6) X3.CGND1 X3.CGND2 X3.CGND3 X3.CGND4 X3.CGND5 X3.CGND6 X4.9(CG1) X4.10(CG2) X4.11(CG3) X4.12(CG4) X5.S1(A:SHLD) X5.S2(A:SHLD) X5.S3(A:SHLD) X5.S4(A:SHLD) X5.S5(B:CG1) X5.S6(B:CG2) X5.S7(B:CG3) X5.S8(B:CG4) X6.20(MTG1) X6.21(MTG2) X6.22(MTG3) X6.22_B(MTG3) X6.23(MTG4) X6.23_B(MTG4)
CLK_25M: TP17.TP U9.23(CLK_25M)
CLKOUT2: C2.2 J4.18(EMU3) J6.41 R3.2 R7.2
DCAN1_RX/TPM_GPIO2: J12.1 U1.C13(C:UART0_RTSN) U16.4(PP/GPIO)
DCAN1_TX/TPM_GPIO1: J12.2 U1.C12(C:UART0_CTSN) U16.3(GPIO-EXPRESS-00)
DVI_+5V: FB6.2 R147.2 R148.2 X6.10(+5V)
EEPROM_WP: J1.1 U1.M2(A:EEPROM_WP)
EHRPWM1A: J6.14 U1.P12(C:GPMC_A2)
EHRPWM1B: J6.16 U1.T13(C:GPMC_A3)
EHRPWM2A: J5.19 U1.T4(C:GPMC_AD8)
EHRPWM2B: J5.13 U1.P5(C:GPMC_AD9)
EMMC_RSTN: R19.2 R52.1 U7.J1(D:NC) U7.J2(D:NC) U7.J3(D:NC) U7.K5(A:RST#)
EMMC_VCCI: C13.2 U7.C1(B:NC) U7.C2(A:VDDI)
ETH_AVDDL: C66.1 C67.1 C68.1 FB2.1 U9.6(AVDDL) U9.11(AVDDL) U9.17(AVDDL)
ETH_DVDDL: C70.1 C71.1 C72.1 FB2.2 L1.P$2 U9.38(DVDDL)
ETH_INT: R142.1 R144.1 U9.20(INT)
ETH_LX: L1.P$1 U9.2(LX)
ETH_VDDIO: C64.1 C65.1 R104.1 U9.8(VDDH_REG) U9.27(VDDIO_REG)
FLASH_EN: J11.2 R155.1 U1.J14(D:RMII1_REF_CLK) U18.D2(A) U19.D2(A) U20.D2(A) U24.D2(A)
GND: C1.1 C2.1 C3.2 C6.1 C11.- C13.1 C14.2 C15.2 C16.1 C17.1 C18.1 C19.1 C20.1 C21.2 C22.2 C23.2 C24.2 C25.2 C26.2 C27.2 C28.2 C29.2 C30.2 C31.2 C32.2 C33.2 C34.2 C35.2 C36.2 C37.2 C38.2 C39.2 C40.2 C41.2 C42.2 C43.2 C44.2 C45.2 C46.2 C47.2 C48.2 C49.2 C50.2 C51.2 C52.2 C53.2 C54.2 C55.2 C56.2 C57.2 C58.2 C59.2 C60.2 C61.2 C62.2 C63.2 C64.2 C65.2 C66.2 C67.2 C68.2 C69.- C70.2 C71.2 C72.2 C73.2 C74.2 C75.2 C76.2 C77.2 C78.2 C79.2 C85.2 C86.2 C87.2 C88.2 C89.2 C90.1 C91.2 C92.2 C93.2 C94.2 C95.2 C96.2 C97.2 C98.2 C99.2 C100.2 C101.2 D2.A D8.3(GND1) D8.8(GND2) D9.3(GND1) D9.8(GND2) J1.2 J2.2 J3.1 J4.4(TDIS) J4.8(GND1) J4.10(GND2) J4.12(GND3) J4.16(GND4) J4.20(GND5) J5.1 J5.2 J6.1 J6.2 J6.43 J6.44 J6.45 J6.46 J7.2 J10.1 J14.2 J14.2_B R1.2 R11.2 R16.1 R18.1 R26.2 R27.1 R34.1 R35.2 R36.2 R37.2 R38.2 R39.1 R53.1 R54.1 R55.1 R56.1 R57.1 R58.1 R59.1 R60.1 R61.1 R62.1 R63.1 R64.1 R65.1 R66.1 R67.1 R68.1 R97.1 R99.1 R100.2 R101.2 R103.1 R105.1 R106.1 R107.1 R109.1 R111.1 R112.1 R113.1 R115.2 R118.1 R128.1 R136.1 R141.1 R155.2 R168.2 S1.2 S1.4 S2.1 S2.3 S3.2 S3.4 TP8.P$1(TP) U1.D8(E:DGND) U1.D9(E:DGND) U1.E5(E:DGND) U1.E6(E:DGND) U1.E7(E:DGND) U1.E8(E:DGND) U1.E9(E:DGND) U1.E10(E:DGND) U1.E11(E:DGND) U1.E12(E:DGND) U1.F5(E:DGND) U1.F12(E:DGND) U1.G5(E:DGND) U1.G12(E:DGND) U1.H4(E:DGND) U1.H5(E:DGND) U1.H12(E:DGND) U1.H13(E:DGND) U1.J4(E:DGND) U1.J5(E:DGND) U1.J12(E:DGND) U1.J13(E:DGND) U1.K5(E:DGND) U1.K12(E:DGND) U1.L5(E:DGND) U1.L12(E:DGND) U1.M5(E:DGND) U1.M6(E:DGND) U1.M7(E:DGND) U1.M8(E:DGND) U1.M9(E:DGND) U1.M10(E:DGND) U1.M11(E:DGND) U1.M12(E:DGND) U1.N8(E:DGND) U1.N9(E:DGND) U2.4(GND) U3.3(GND) U4.5(GND) U6.1(*1OE) U6.4(GND) U7.A6(A:VSS1) U7.C4(A:VSSQ1) U7.D3(C:NC) U7.E2(C:NC) U7.E7(A:VSS2) U7.F1(C:NC) U7.G5(A:VSS3) U7.H10(A:VSS4) U7.J5(A:VSS5) U7.K8(A:VSS6) U7.N1(E:NC) U7.N2(A:VSSQ2) U7.N5(A:VSSQ3) U7.P4(A:VSSQ4) U7.P6(A:VSSQ5) U8.37(VSS) U9.41(PAD) U10.8(VPB1) U10.9(VPB0) U10.16(VPC2) U10.17(VPC1) U10.18(VPC0) U10.19(VPP) U10.53(A0_I2C) U10.54(A1_I2C) U10.61(VPA2) U10.62(VPA1) U10.63(VPA0) U10.65(PAD) U11.4(GND) U12.4(GND) U13.4(GND) U14.4(GND) U15.1(GND) U15.TH(PAD) U16.2(GND) U16.5(TESTL) U16.6(XTAMPER) U16.9(GND) U16.18(PIRQ#) U16.19(ATEST) U16.20(TWI_WAKEUP#) U16.21(ATEST) U16.23(GND) U16.24(ATEST) U16.32(GND) U17.A4(GND) U17.B4(ADD) U18.B1(INH) U18.C1(GND) U18.D1(GND) U19.B1(INH) U19.C1(GND) U19.D1(GND) U20.B1(INH) U20.C1(GND) U20.D1(GND) U21.4(VSS) U22.3(RESERVED) U22.5(SDO/SA0) U22.8(GND) U22.9(GND) U23.9(AD0/SDO) U23.18(GND) U23.20(RESV) U24.B1(INH) U24.C1(GND) U24.D1(GND) U25.1(GND) U26.6(GND) X1.GND X3.6(VSS) X3.GND X4.4(GND) X4.8(GND) X5.1(A:GND) X5.U14(B:GND) X5.U24(B:GND) X6.2(DAT1_SMTG3) X6.5(CLK_S) X6.8(DDC/CEC-GND) X6.13(DAT0_S) X6.16(DAT2_S) Y3.2(GND) Y5.2(GND)
GPIO0_7: J6.42 R2.2 R9.2
GPIO0_7SRC: R2.1 U1.C5(C:ECAP0_IN_PWM0_OUT)
GPIO0_26: J5.14 U1.R5(C:GPMC_AD10)
GPIO0_27: J5.17 U1.T5(C:GPMC_AD11)
GPIO1_12: J5.12 U1.P6(C:GPMC_AD12)
GPIO1_13: J5.11 U1.R6(C:GPMC_AD13)
GPIO1_14: J5.16 U1.T6(C:GPMC_AD14)
GPIO1_15: J5.15 U1.P7(C:GPMC_AD15)
GPIO1_16: J6.15 R14.2 R23.2
GPIO1_17: J6.23 U1.R12(C:GPMC_A1)
GPIO1_28: J6.12 U1.N14(C:GPMC_BEN1)
GPIO1_29: J5.26 U1.P3(C:GPMC_CSN0)
GPIO2_1: J5.18 U1.T7(C:GPMC_CLK)
GPIO3_18: R9.1 U1.A3(C:MCASP0_ACLKR)
GPIO3_19: J6.27 U1.B3(C:MCASP0_FSR)
GPIO3_20: R7.1 U1.C3(C:MCASP0_AXR1)
GPIO3_21: J6.25 R114.2 U1.C4(C:MCASP0_AHCLKX)
HDMI_CEC: D11.C(CATHODE) U10.30(CEC) X6.12(CEC)
HDMI_CEC_D: D11.A(ANODE) R140.2
HDMI_CLK_INH: J7.1 R110.1 Y3.1(INH#)
HDMI_DSCL: R147.1 U10.33(DSCL) X6.11(SCL)
HDMI_DSDA: R148.1 U10.32(DSDA) X6.9(SDA)
HDMI_HPD: U10.31(HPD) X6.19(HPLG)
HDMI_INT: R130.1 U1.T15(C:GPMC_A9) U10.50(INT)
HDMI_SWING: R136.2 U10.34(EXT_SWING)
HDMI_TX0+: D9.5(TMDS.CH2-) D9.6(NC1) U10.40(TX0+) X6.15(DAT0+)
HDMI_TX0-: D9.4(TMDS.CH2+) D9.7(NC2) U10.39(TX0-) X6.14(DAT0-)
HDMI_TX1+: D8.2(TMDS.CH1-) D8.9(NC3) U10.43(TX1+) X6.3(DAT1+)
HDMI_TX1-: D8.1(TMDS.CH1+) D8.10(NC4) U10.42(TX1-) X6.4(DAT1-)
HDMI_TX2+: D8.5(TMDS.CH2-) D8.6(NC1) U10.45(TX2+) X6.18(DAT2+)
HDMI_TX2-: D8.4(TMDS.CH2+) D8.7(NC2) U10.44(TX2-) X6.17(DAT2-)
HDMI_TXC+: D9.2(TMDS.CH1-) D9.9(NC3) U10.38(TXC+) X6.6(CLK+)
HDMI_TXC-: D9.1(TMDS.CH1+) D9.10(NC4) U10.37(TXC-) X6.7(CLK-)
HDMICLK_DISN: U1.T16(C:GPMC_A11) Y5.1(INH#)
I2C0_SCL: J15.1 R12.1 U1.C10(A:I2C0_SCL) U1.D10(A:PMIC_SCL) U10.52(CSCL) U16.29(SM_CLK) U17.D4(SCL) U22.2(SCL/SPC) U25.6(SCL2)
I2C0_SCL_1P8V: R163.1 U23.23(SCL/SCLK) U25.3(SCL1)
I2C0_SDA: J15.2 R13.1 U1.C11(A:I2C0_SDA) U1.D11(A:PMIC_SDA) U10.51(CSDA) U16.30(SM_DAT) U17.C4(SDA) U22.4(SDA/SDI/SDO) U25.5(SDA2)
I2C0_SDA_1P8V: R164.1 U23.24(SDA/SDI) U25.4(SDA1)
I2C1_SCL: J6.17 R154.2 U18.B2(Y1)
I2C1_SCL_COMB: R154.1 U1.A14(C:SPI0_CS0) U18.A1(COM)
I2C1_SDA: J6.18 R159.2 U20.B2(Y1)
I2C1_SDA_COMB: R159.1 U1.B14(C:SPI0_D1) U20.A1(COM)
I2C2_SCL: J6.19 U1.A10(C:UART1_RTSN)
I2C2_SDA: J6.20 U1.B10(C:UART1_CTSN)
IMU_INT: U1.E15(D:MII1_RX_ER) U23.12(INT1)
JTAG_EMU0: J4.13(EMU0) R40.1 U1.E2(B:EMU0)
JTAG_EMU1: J4.14(EMU1) R41.1 U1.E3(B:EMU1)
JTAG_TCK: J4.9(TCKRTN) J4.11(TCK) U1.D1(B:TCK)
JTAG_TDI: J4.3(TDI) U1.C1(B:TDI)
JTAG_TDO: J4.7(TDO) U1.C2(B:TDO)
JTAG_TMS: J4.1(TMS) U1.D2(B:TMS)
JTAG_TRSTN: J4.2(TRSTN) R39.2 U1.D3(B:TRSTN)
LCD_DATA0: C38.1 J5.45 R68.2 R85.1 U1.G3(D:LCD_DATA0) U10.15(VPC3)
LCD_DATA1: C37.1 J5.46 R67.2 R84.1 U1.G2(D:LCD_DATA1) U10.13(VPC4)
LCD_DATA2: C36.1 J5.43 R66.2 R69.1 R83.1 U1.G1(D:LCD_DATA2) U10.12(VPC5)
LCD_DATA3: C35.1 J5.44 R65.2 R82.1 U1.H3(D:LCD_DATA3) U10.11(VPC6)
LCD_DATA4: C34.1 J5.41 R64.2 R81.1 U1.H2(D:LCD_DATA4) U10.10(VPC7)
LCD_DATA5: C28.1 J5.42 R63.2 R80.1 U1.H1(D:LCD_DATA5) U10.7(VPB2)
LCD_DATA6: C27.1 J5.39 R62.2 R79.1 U1.J3(D:LCD_DATA6) U10.6(VPB3)
LCD_DATA7: C26.1 J5.40 R61.2 R78.1 U1.J2(D:LCD_DATA7) U10.3(VPB4)
LCD_DATA8: C25.1 J5.37 R60.2 R77.1 U1.J1(D:LCD_DATA8) U10.2(VPB5)
LCD_DATA9: C24.1 J5.38 R59.2 R76.1 U1.K3(D:LCD_DATA9) U10.1(VPB6)
LCD_DATA10: C23.1 J5.36 R58.2 R75.1 U1.K2(D:LCD_DATA10) U10.64(VPB7)
LCD_DATA11: C33.1 J5.34 R57.2 R74.1 U1.K1(D:LCD_DATA11) U10.60(VPA3)
LCD_DATA12: C32.1 J5.35 R56.2 R73.1 U1.L3(D:LCD_DATA12) U10.59(VPA4)
LCD_DATA13: C31.1 J5.33 R55.2 R72.1 U1.L2(D:LCD_DATA13) U10.58(VPA5)
LCD_DATA14: C30.1 J5.31 R54.2 R71.1 U1.L1(D:LCD_DATA14) U10.57(VPA6)
LCD_DATA15: C29.1 J5.32 R53.2 R70.1 U1.M3(D:LCD_DATA15) U10.56(VPA7)
LCD_DE: J5.30 R28.2 U10.20(DE/VREF)
LCD_HSYNC: J5.29 R29.2 U10.22(HSYNC/VREF)
LCD_PCLK: J5.28 R31.2 U10.4(PCLK)
LCD_VSYNC: J5.27 R30.2 U10.21(VSYNC/VREF)
LDO_PGOOD: TP22.TP U1.N4(A:PMIC_LDO_PGOOD) U1.N5(A:RTC_PWRONRSTN)
LED_10_100: C45.1 R93.1 U9.24(LED_10_100) X5.13(A:D13)
LED_1000: C44.1 R96.2 U9.22(LED_1000) X5.15(A:D15)
LED_ACT: C46.1 R104.2 U9.21(LED_ACT) X5.11(A:D11)
MDC: R139.1 U9.40(MDC)
MDIO: R138.1 R145.2 U9.39(MDIO)
MDIO_CLK: R139.2 U1.D13(D:MDC)
MDIO_DATA: R138.2 U1.E13(D:MDIO)
MII1_COL: R142.2 U1.F15(D:MII1_COL)
MII1_RXCLK: R127.2 U1.E16(D:MII1_RX_CLK)
MII1_RXD0: R125.2 U1.E14(D:MII1_RXD0)
MII1_RXD1: R122.2 U1.D16(D:MII1_RXD1)
MII1_RXD2: R121.2 U1.D15(D:MII1_RXD2)
MII1_RXD3: R120.2 U1.D14(D:MII1_RXD3)
MII1_RXDV: R126.2 U1.F16(D:MII1_RX_DV)
MII1_TXCLK: R135.2 U1.H16(D:MII1_TX_CLK)
MII1_TXD0: R133.2 U1.H15(D:MII1_TXD0)
MII1_TXD1: R132.2 U1.H14(D:MII1_TXD1)
MII1_TXD2: R131.2 U1.G16(D:MII1_TXD2)
MII1_TXD3: R129.2 U1.G15(D:MII1_TXD3)
MII1_TXEN: R134.2 U1.G14(D:MII1_TX_EN)
MMC0_CD: J4.19(EMU4) R92.1 U1.C14(C:SPI0_CS1) X3.CD(CD#)
MMC0_CLK: R88.1 U1.B15(C:MMC0_CLK) X3.5(CLK)
MMC0_CMD: R87.1 U1.B16(C:MMC0_CMD) X3.3(CMD/DI)
MMC0_DAT0: R89.1 U1.A16(C:MMC0_DAT0) X3.7(DAT0/DO)
MMC0_DAT1: R90.1 U1.A15(C:MMC0_DAT1) X3.8(DAT1)
MMC0_DAT2: R86.1 U1.C16(C:MMC0_DAT2) X3.1(DAT2)
MMC0_DAT3: R91.1 U1.C15(C:MMC0_DAT3) X3.2(DAT3/CS)
MMC1_CLK: J5.21 R51.1 U1.P2(C:GPMC_CSN1) U7.M6(A:CLK) U7.N7(E:NC) U7.P8(E:NC)
MMC1_CMD: J5.20 R50.1 U1.P1(C:GPMC_CSN2) U7.M5(A:CMD) U7.N6(E:NC) U7.P7(E:NC)
MMC1_DAT0: J5.25 R42.1 U1.R3(C:GPMC_AD0) U7.A3(A:DAT0)
MMC1_DAT1: J5.24 R43.1 U1.R2(C:GPMC_AD1) U7.A4(A:DAT1)
MMC1_DAT2: J5.5 R44.1 U1.R1(C:GPMC_AD2) U7.A5(A:DAT2)
MMC1_DAT3: J5.6 R45.1 U1.T3(C:GPMC_AD3) U7.A1(B:NC) U7.B2(A:DAT3)
MMC1_DAT4: J5.23 R46.1 U1.T2(C:GPMC_AD4) U7.A2(B:NC) U7.B3(A:DAT4)
MMC1_DAT5: J5.22 R47.1 U1.T1(C:GPMC_AD5) U7.B4(A:DAT5) U7.C3(B:NC) U7.D2(C:NC) U7.E1(C:NC)
MMC1_DAT6: J5.3 R48.1 U1.P4(C:GPMC_AD6) U7.A10(B:NC) U7.B5(A:DAT6) U7.B9(B:NC) U7.C5(B:NC) U7.C8(B:NC)
MMC1_DAT7: J5.4 R49.1 U1.R4(C:GPMC_AD7) U7.A8(B:NC) U7.B6(A:DAT7) U7.B7(B:NC)
MON_OUT: C97.1 R167.1 U4.1(VOUT)
N$1: R10.1 X1.VBUS
N$2: D7.2(C) R38.1
N$3: R69.2 S3.1 S3.3
N$5: C100.1 C101.1 U8.34(NC)
N$6: TP1.TP U1.F4(F:VDDS_DDR)
N$7: R8.1 U8.5(NC)
N$8: D1.2(C) R26.1
N$9: R15.2 R20.1 U5.1(REF)
N$10: Q1.B R21.1 U5.2(CATHODE)
N$11: D6.2(C) R37.1
N$13: D5.2(C) R36.1
N$14: TP9.TP U8.13(OCS1_N)
N$15: D4.2(C) R35.1
N$16: R102.1 Y3.3(OUT)
N$17: TP10.TP U8.17(OCS2_N)
N$18: TP2.TP U1.G4(F:VDD_CORE)
N$19: TP3.TP U1.F13(F:VDD_MPU)
N$20: R3.1 U1.B4(C:XDMA_EVENT_INTR1)
N$21: TP4.TP U1.G13(F:VDDS_PLL)
N$22: R4.1 U1.A4(C:XDMA_EVENT_INTR0)
N$23: R161.2 U21.3(W#)
N$24: R11.1 R166.2 U8.27(VBUS_DET)
N$25: R160.2 U21.7(HOLD#)
N$26: R19.1 U1.R13(C:GPMC_A4)
N$28: J10.4 R153.1
N$29: J10.6 R152.1
N$30: C96.1 U4.3(C_T)
N$31: J10.8 R151.1
N$32: J10.10 R150.1
N$33: R1.1 U1.M16(A:RTC_KALDO_ENN)
N$34: Q2.B Q2.C R149.1
N$35: J11.1 R157.2
N$36: R146.2 TP25.P$1(TP) U9.1(RSTN)
N$38: C91.1 U23.10(REGOUT)
N$42: R114.1 Y5.3(OUT)
N$47: R100.1 U8.35(RBIAS)
N$48: C42.1 C99.1 U8.14(VDDCR12)
N$49: R118.2 U10.49(TEST)
N$53: R23.1 U1.T12(C:GPMC_A0)
N$57: D10.1(A) U8.11(LED0)
N$58: R14.1 U1.R7(C:GPMC_CSN3)
N$59: D10.2(C) R128.2
N$64: R123.2 X5.12(A:D12)
N$65: R124.2 X5.14(A:D14)
N$70: R31.1 U1.F1(D:LCD_PCLK)
N$72: R30.1 U1.F3(D:LCD_VSYNC)
N$77: R119.1 U9.4(XTLO)
N$83: R29.1 U1.F2(D:LCD_HSYNC)
N$85: R28.1 U1.E1(D:LCD_AC_BIAS_EN)
NON_REM0: R105.2 TP19.P$1(TP) U8.28(SUSP_IND/NON_REM0)
NON_REM1: J8.1 R103.2 U8.22(SDA/NON_REM1)
OSC0_GND: C7.2 C12.2 U1.N15(B:OSC0_GND)
OSC0_IN: C12.1 R32.2 U1.P16(B:OSC0_IN) Y2.P$2
OSC0_OUT: C7.1 R32.1 U1.N16(B:OSC0_OUT) Y2.P$1
OSC1_GND: C4.2 C5.2 U1.B5(B:OSC1_GND)
OSC1_IN: C5.1 R24.2 U1.A6(B:OSC1_IN) Y1.P$2
OSC1_OUT: C4.1 R24.1 U1.A5(B:OSC1_OUT) Y1.P$1
PHY_XTAL1: C60.1 R117.1 R119.2 Y6.P$2
PHY_XTAL2: R116.1 U9.5(XTLI)
PHYX: C47.1 R116.2 R117.2 Y6.P$1
PMIC_INT: TP24.TP U1.D4(A:EXTINTN) U1.E4(A:PMIC_NINT)
PMIC_MUX_IN: R18.2 R22.1 U1.N13(B:PMIC_MUX_IN)
PMIC_NRESET: J2.1 U1.M13(A:PMIC_NRESET)
PMIC_NWAKEUP: TP23.TP U1.L4(A:PMIC_NWAKEUP) U1.M4(A:EXT_WAKEUP)
PMIC_PGOOD: U1.N12(A:PMIC_PGOOD) U1.P11(A:PWRONRSTN) U3.2(A)
PWR_BUT: J6.9 S2.2 S2.4 U1.T11(A:PMIC_PB_IN)
PWR_EN: TP21.TP U1.N10(A:PMIC_POWER_EN) U1.N11(A:PMIC_PWR_EN)
RBIAS: R115.1 U9.7(RBIAS)
RX_CLK: R94.1 R127.1 U9.31(RX_CLK)
RX_DV: R101.1 R126.1 U9.30(RX_DV)
RXD0: R109.2 R125.1 U9.29(RXD0)
RXD1: R106.2 R122.1 U9.28(RXD1)
RXD2: R98.1 R121.1 U9.26(RXD2)
RXD3: R95.1 R120.1 U9.25(RXD3)
SPI0_CS0: R158.1 TP30.TP U18.C2(Y2) U21.1(S#)
SPI0_D0(MISO): TP29.TP U19.C2(Y2) U21.2(DQ1)
SPI0_D1(MOSI): TP28.TP U20.C2(Y2) U21.5(DQ0)
SPI0_SCLK: TP27.TP U21.6(C) U24.C2(Y2)
SPI1_CS0: J6.28 U1.B1(C:MCASP0_AHCLKR) U10.25(AP1)
SPI1_D0: J6.29 U1.A2(C:MCASP0_FSX) U10.24(AP0)
SPI1_D1: J6.30 U1.B2(C:MCASP0_AXR0)
SPI1_SCLK: J6.31 U1.A1(C:MCASP0_ACLKX) U10.23(ACLK)
SYS_ADC_1P8V: C10.1 J6.32 R33.2 U1.A7(B:SYS_ADC_1P8V)
SYS_RESETN: C14.1 C94.1 J4.15(SRST) J6.10 R5.2 S1.1 S1.3 TP26.P$1(TP) U1.R11(A:WARMRSTN) U3.4(Y) U16.17(LRESET#)
SYS_RTC_1P8V: Q1.C R15.1 TP14.TP U1.K11(A:SYS_RTC_1P8V) U1.L11(A:SYS_RTC_1P8V) U3.5(VCC) U5.3(ANODE)
SYS_VDD1_3P3V: C6.2 C15.1 C16.2 C17.2 C18.2 C19.2 C20.2 C21.1 C22.1 C39.1 C43.1 C48.1 C49.1 C50.1 C51.1 C61.1 C62.1 C63.1 C75.1 C76.1 C79.1 C85.1 C86.1 C87.1 C88.1 C90.2 C92.1 C93.1 FB5.1 J4.5(TVDD) J6.3 J6.4 J10.2 R5.1 R8.2 R12.2 R13.2 R17.2 R22.2 R40.2 R41.2 R42.2 R43.2 R44.2 R45.2 R46.2 R47.2 R48.2 R49.2 R50.2 R51.2 R52.2 R70.2 R71.2 R72.2 R73.2 R74.2 R75.2 R76.2 R77.2 R78.2 R79.2 R80.2 R81.2 R82.2 R83.2 R84.2 R85.2 R86.2 R87.2 R88.2 R89.2 R90.2 R91.2 R92.2 R93.2 R94.2 R95.2 R96.1 R98.2 R110.2 R130.2 R137.1 R140.1 R143.2 R144.2 R145.1 R146.1 R157.1 R158.2 R160.1 R161.1 TP12.TP U1.F6(A:SYS_VDD1_3P3V) U1.F7(A:SYS_VDD1_3P3V) U1.G6(A:SYS_VDD1_3P3V) U1.G7(A:SYS_VDD1_3P3V) U6.7(2OE) U6.8(VCC) U7.A9(B:NC) U7.B8(B:NC) U7.C6(A:VCCQ1) U7.C7(B:NC) U7.E6(A:VCC1) U7.F5(A:VCC2) U7.J10(A:VCC3) U7.K9(A:VCC4) U7.M4(A:VCCQ2) U7.N4(A:VCCQ3) U7.P1(E:NC) U7.P2(E:NC) U7.P3(A:VCCQ4) U7.P5(A:VCCQ5) U8.10(VDDA33) U8.15(VDD33) U8.23(VDD33) U8.29(VDDA33) U8.36(VDDA33) U9.3(VDD33) U16.1(VCC) U16.8(VCC) U16.22(VCC) U17.D3(V+) U18.A2(VCC) U19.A2(VCC) U20.A2(VCC) U21.8(VCC) U22.1(VDD_IO) U22.6(CS) U22.10(VDD) U23.13(VDD) U24.A2(VCC) X3.4(VDD) Y3.4(VCC) Y5.4(VCC)
SYS_VDD2_3P3V: D1.1(A) TP13.TP U1.F11(A:SYS_VDD2_3P3V) U1.G11(A:SYS_VDD2_3P3V)
SYS_VDD3_3P3V: Q1.E R20.2 R21.2 TP16.TP U1.F8(A:SYS_VDD3_3P3V) U1.F9(A:VDDSHV4) U1.G8(A:SYS_VDD3_3P3V) U1.G9(A:VDDSHV5) U1.H7(A:SYS_VDD3_3P3V) U1.H8(A:SYS_VDD3_3P3V) U1.H9(A:VDDSHV6) U1.J7(A:SYS_VDD3_3P3V) U1.J8(A:SYS_VDD3_3P3V) U1.J9(A:VDDSHV1) U1.K8(A:SYS_VDD3_3P3V) U1.K9(A:VDDSHV2) U1.L8(A:SYS_VDD3_3P3V) U1.L9(A:VDDSHV3)
SYS_VDD_1P8V: C89.1 FB1.2 R163.2 R164.2 TP15.TP U1.F10(A:SYS_VDD_1P8V) U1.G10(A:SYS_VDD_1P8V) U1.H10(A:SYS_VDD_1P8V) U1.H11(A:SYS_VDD_1P8V) U1.J10(A:SYS_VDD_1P8V) U1.J11(A:SYS_VDD_1P8V) U1.K10(A:SYS_VDD_1P8V) U1.L10(A:SYS_VDD_1P8V) U23.8(VDDIO) U23.22(NCS) U25.2(VREF1)
SYS_VOUT: C69.+ FB6.1 J6.7 J6.8 TP11.TP U1.K6(A:SYS_VOUT) U1.K7(A:SYS_VOUT) U1.L6(A:SYS_VOUT) U1.L7(A:SYS_VOUT) U15.2(IN1) U15.3(IN2)
TEMP_D1+: C84.1 R153.2 U17.A1(D1+)
TEMP_D2+: C83.1 R152.2 U17.B1(D2+)
TEMP_D3+: C82.1 R151.2 U17.C1(D3+)
TEMP_D4+: C81.1 R150.2 U17.D1(D4+)
TEMP_D8+: C80.1 R149.2 U17.D2(D8+)
TEMP_D-: C80.2 C81.2 C82.2 C83.2 C84.2 J10.3 J10.5 J10.7 J10.9 Q2.E U17.A2(D5+) U17.A3(D-) U17.B2(D6+) U17.C2(D7+)
TEMP_SENSE: TP7.P$1(TP) U1.N6(A:PMIC_TS)
TIMER4: J5.7 U1.M1(C:GPMC_ADVN_ALE)
TIMER5: J5.9 U1.N3(C:GPMC_BEN0_CLE)
TIMER6: J5.10 U1.N2(C:GPMC_WEN)
TIMER7: J5.8 U1.N1(C:GPMC_OEN_REN)
TPM_GPIO0: U1.F14(D:MII1_CRS) U16.12(GPIO)
TRXN0: U9.10(TRXN0) X5.3(A:TRD1-)
TRXN1: U9.13(TRXN1) X5.5(A:TRD2-)
TRXN2: U9.16(TRXN2) X5.8(A:TRD3-)
TRXN3: U9.19(TRXN3) X5.10(A:TRD4-)
TRXP0: U9.9(TRXP0) X5.2(A:TRD1+)
TRXP1: U9.12(TRXP1) X5.4(A:TRD2+)
TRXP2: U9.15(TRXP2) X5.7(A:TRD3+)
TRXP3: U9.18(TRXP3) X5.9(A:TRD4+)
TX_CLK: R135.1 U9.33(GTX_CLK)
TX_EN: R134.1 U9.32(TX_EN)
TXD0: R133.1 U9.34(TXD0)
TXD1: R132.1 U9.35(TXD1)
TXD2: R131.1 U9.36(TXD2)
TXD3: R129.1 U9.37(TXD3)
UART0_RX: U1.A12(C:UART0_RXD) U6.6(1Y)
UART0_TX: U1.B12(C:UART0_TXD) U6.5(2A)
UART1_RXD: J6.26 U1.A11(C:UART1_RXD)
UART1_TXD: J6.24 U1.B11(C:UART1_TXD)
UART2_RXD: J6.22 R162.2 U24.B2(Y1)
UART2_RXD_COMB: R162.1 U1.A13(C:SPI0_SCLK) U24.A1(COM)
UART2_TXD: J6.21 R156.2 U19.B2(Y1)
UART2_TXD_COMB: R156.1 U1.B13(C:SPI0_D0) U19.A1(COM)
UART4_RXD: J6.11 U1.P15(C:GPMC_WAIT0)
UART4_TXD: J6.13 U1.R16(C:GPMC_WPN)
USB0_DM: U1.K16(B:USB0_DM) U2.1(D-) X1.D-
USB0_DP: U1.K15(B:USB0_DP) U2.2(D+) X1.D+
USB0_ID: U1.K14(B:USB0_ID) U2.3(ID) X1.ID
USB1_DM: U1.L16(B:USB1_DM) U8.30(USBUP_DM)
USB1_DP: U1.L15(B:USB1_DP) U8.31(USBUP_DP)
USB1_DRVVBUS: R141.2 U1.M14(B:USB1_DRVVBUS) U15.4(EN)
USB1_ID: R16.2 U1.L14(B:USB1_ID)
USB1_OCN: R143.1 U1.R15(C:GPMC_A10) U15.5(!OC)
USB1_PWR: FB3.2 FB4.1 U15.6(OUT1) U15.7(OUT2) U15.8(OUT3)
USB1_VBUS: FB3.1 U1.M15(B:USB1_VBUS)
USB_OSC1: C41.1 R108.2 U8.33(XTAL1) Y4.P$2
USB_OSC2: C40.1 R108.1 U8.32(XTAL2) Y4.P$1
USB_RESET: R137.2 TP18.P$1(TP) U8.26(RESET_N)
USB_UART_RX: J9.1 U8.19(OCS3_N)
USB_UART_TX: J9.2 U8.21(OCS4_N)
USBHUB0_DM: U8.1(USBDN1_DM) U11.2(D-) X5.U22(B:D-)
USBHUB0_DP: U8.2(USBDN1_DP) U11.1(D+) X5.U23(B:D+)
USBHUB1_DM: U8.3(USBDN2_DM) U12.2(D-) X5.U12(B:D-)
USBHUB1_DP: U8.4(USBDN2_DP) U12.1(D+) X5.U13(B:D+)
USBHUB2_DM: U8.6(USBDN3_DM) U13.2(D-) X4.6(D-)
USBHUB2_DP: U8.7(USBDN3_DP) U13.1(D+) X4.7(D+)
USBHUB3_DM: U8.8(USBDN4_DM) U14.2(D-) X4.2(D-)
USBHUB3_DP: U8.9(USBDN4_DP) U14.1(D+) X4.3(D+)
USR0: D7.1(A) U1.P13(C:GPMC_A5)
USR1: D6.1(A) U1.T14(C:GPMC_A6)
USR2: D5.1(A) U1.R14(C:GPMC_A7)
USR3: D4.1(A) U1.P14(C:GPMC_A8)
VBUS: C73.1 C74.1 FB4.2 R166.1 U11.6(VBUS) U12.6(VBUS) U13.6(VBUS) U14.6(VBUS) X4.1(VBUS) X4.5(VBUS) X5.U11(B:VBUS) X5.U21(B:VBUS)
VDD_5V: C95.1 C98.1 J6.5 J6.6 R168.1 U1.P10(A:VIN_AC) U1.R10(A:VIN_AC) U1.T10(A:VIN_AC) U26.5(VOUT) U26.8(VOUT)
VDD_BAT: R165.2 TP5.P$1(TP) U1.P8(A:VIN_BAT) U1.R8(A:VIN_BAT) U1.T8(A:VIN_BAT)
VDD_ETH_PHY: C77.1 C78.1 FB5.2 R123.1 R124.1 U9.14(AVDD33)
VDD_HDMI_1P8V: C52.1 C53.1 C54.1 C55.1 C56.1 C57.1 C58.1 C59.1 FB1.1 U10.5(VDDDC0(1.8V)) U10.14(VDDIOA(1.8V)) U10.29(VDDDC1(1.8V)) U10.35(VDDA0(1.8V)) U10.36(VDDA1(TX)(1.8V)) U10.41(VDDA2(TX)(1.8V)) U10.46(VDDA3(TX)(1.8V)) U10.47(VDDA(PLL0)(1.8V)) U10.48(VDDA(PLL1)(1.8V)) U10.55(VDDIOB(1.8V))
VDD_USB_5V: C3.1 R10.2 U1.J16(B:USB0_VBUS) U1.P9(A:VIN_USB) U1.R9(A:VIN_USB) U1.T9(A:VIN_USB) U2.6(VBUS)
VIN: C11.+ D2.C F1.2 R6.2 U4.2(SUB) U4.4(VDD) U26.1(VIN) U26.3(VBIAS) U26.4(VIN)
VIN_CTL: R6.1 R167.2 U26.2(ON)
VIN_PREDIODE: D3.A J14.1 J14.1_B
VIN_PREFUSE: D3.C F1.1
VREF2: R17.1 U25.7(VREF2) U25.8(EN)
VREFN: R25.1 U1.B9(B:VREFN)
VREFP: C8.1 C9.1 R33.1 U1.B7(B:VREFP)
XDMA_EVENT_INTR0: C1.2 J4.17(EMU2) R4.2
Unconnected: FUD1.P$1 FUD2.P$1 FUD3.P$1 FUD4.P$1 FUD5.P$1 FUD6.P$1 J3.2 J3.3 J3.6 J4.6(NC) J14.3 J14.3_B U1.D5(F:CAP_VDD_RTC) U1.D12(F:NC) U1.H6(F:VPP) U1.J6(F:NC) U1.J15(B:USB0_DRVVBUS) U1.K4(F:NC) U1.K13(B:USB0_CE) U1.L13(B:USB1_CE) U2.5(N.C.) U3.1(NC) U7.A7(A:RFU) U7.A11(B:NC) U7.A12(B:NC) U7.A13(B:NC) U7.A14(B:NC) U7.B1(B:NC) U7.B10(B:NC) U7.B11(B:NC) U7.B12(B:NC) U7.B13(B:NC) U7.B14(B:NC) U7.C9(B:NC) U7.C10(B:NC) U7.C11(B:NC) U7.C12(B:NC) U7.C13(B:NC) U7.C14(C:NC) U7.D1(C:NC) U7.D4(C:NC) U7.D12(C:NC) U7.D13(C:NC) U7.D14(C:NC) U7.E3(C:NC) U7.E5(A:RFU) U7.E8(A:VSF) U7.E9(A:VSF) U7.E10(A:VSF) U7.E12(C:NC) U7.E13(C:NC) U7.E14(C:NC) U7.F2(C:NC) U7.F3(C:NC) U7.F10(A:VSF) U7.F12(C:NC) U7.F13(C:NC) U7.F14(C:NC) U7.G1(C:NC) U7.G2(C:NC) U7.G3(C:NC) U7.G10(A:VSF) U7.G12(C:NC) U7.G13(C:NC) U7.G14(C:NC) U7.H1(C:NC) U7.H2(C:NC) U7.H3(D:NC) U7.H5(A:DS) U7.H12(D:NC) U7.H13(D:NC) U7.H14(D:NC) U7.J12(D:NC) U7.J13(D:NC) U7.J14(D:NC) U7.K1(D:NC) U7.K2(D:NC) U7.K3(D:NC) U7.K6(A:RFU) U7.K7(A:RFU) U7.K10(A:VSF) U7.K12(D:NC) U7.K13(D:NC) U7.K14(D:NC) U7.L1(D:NC) U7.L2(D:NC) U7.L3(D:NC) U7.L12(D:NC) U7.L13(D:NC) U7.L14(D:NC) U7.M1(D:NC) U7.M2(D:NC) U7.M3(D:NC) U7.M7(D:NC) U7.M8(D:NC) U7.M9(D:NC) U7.M10(E:NC) U7.M11(E:NC) U7.M12(E:NC) U7.M13(E:NC) U7.M14(E:NC) U7.N3(E:NC) U7.N8(E:NC) U7.N9(E:NC) U7.N10(E:NC) U7.N11(E:NC) U7.N12(E:NC) U7.N13(E:NC) U7.N14(E:NC) U7.P9(E:NC) U7.P10(A:VSF) U7.P11(E:NC) U7.P12(E:NC) U7.P13(E:NC) U7.P14(E:NC) U10.26(AP2) U10.28(AP3) U11.3(ID) U11.5(N.C.) U12.3(ID) U12.5(N.C.) U13.3(ID) U13.5(N.C.) U14.3(ID) U14.5(N.C.) U16.7(NC) U16.10(NC) U16.11(NC) U16.13(NC) U16.14(NC) U16.15(NC) U16.16(NC) U16.25(NC) U16.26(NC) U16.27(NC) U16.28(NC) U16.31(NC) U16.33(PAD) U17.B3(THERM#) U17.C3(THERM2#) U21.PAD U22.7(INT_DRDY) U23.1(NC) U23.2(NC) U23.3(NC) U23.4(NC) U23.5(NC) U23.6(NC) U23.7(AUX_CL) U23.11(FSYNC) U23.14(NC) U23.15(NC) U23.16(NC) U23.17(NC) U23.19(RESV) U23.21(AUX_DA) U26.7(CT) X5.6(A:VCC) X6.1(NC)

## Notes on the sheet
- 9-axis IMU | Barometer | Secure NOR Boot Flash | Notes
- I2C Address: 0x68 | I2C Address: 0x5C | Switch bypass
- Rev 4:  
      1) Initial Production Release.
- 2018/05/14 (schematic only update):  
    1) Added note to calculate capacitance for C7 and C21
    2) Added complete part number of APX811
- There are many footprint compatible
  (8-WSON) parts for the NOR flash
  if the listed part is not available.
- 2018/11/15 (schematic only update):  
    1) Upated component values to match BOM / remove un-needed tolerances / voltages
    2) Added notes on I2C0 pull-ups and TPD4S012
- 2019/03/25 (schematic only update):  
    1) Added notes on USBx_VBUS and eMMC reset
    2) Added I2C addresses for all I2C components
- Switch bypass
- 2021/03/08:  
    1) Updated U23 - replaced IMU-9250 (obsolete) with ICM-20948
    2) Added U25 for 3.3V <-> 1.8V voltage translation for U23
    3) Shorted pin 20 of U23 to GND
    4) R158 pulled up to SYS_VDD1_3P3V
    5) Updated D8 & D9 - replaced IP4283CZ10 with TPD4E05U06
    6) eMMC routing updated to be compatible with JEDEC spec v5.x
    7) Updated Octavo Logo to v2
    8) Soldermask polygon of U17, U18, U19, U20, U24 updated
    9) Component values of R8, R157 updated
    10) U7 & U16 alternate part numbers added under notes in Sch
    11) 0 ohm jumper (R165) added between VIN_BAT & PMIC_BAT_SENSE
    12) Eth Phy strapping improved - values of R123, R124 updated, LED_ACT pull up moved to ETH_VDDIO
    13) Reset Supervisor circuit updated to mitigate PMIC lockup due to VIN Brownout fault. 
      See Solution3 of http://www.ti.com/lit/an/slva901/slva901.pdf
    14) 2 pin jumper J12 added for DCAN interface. Silkscreen improved
    15) Barometer U22 updated due to part sourcing issues
    16) MPN and package names updated
    17) Silk screen refined
    18) Added R168 to be used as a bleed resistor in case brownout load switch does not have QOD
- By default, if jumper is not 
  populated, then the flash is 
  disconnected from the OSD3358.  
  If jumper is populated, the 
  stronger pull-up will connect 
  the flash by default.
- To be pin compatible with the Cape headers, we need to be able to
  connect or disconnect the flash memory from the OSD335x-SM.  This circuit 
  accomplishes that.  When pin S# on the flash is low, the flash will ignore 
  all other inputs.  Therefore, there is a 100K pull-down on SPI0_CS0 that 
  will pull that pin low when the flash is disconnected.  Given that I2C1 
  pins might have pull-up resistors on a cape or the UART2 pins could be 
  connected, we need to use 2:1 analog switches to connect or disconnect the 
  flash.
- Switch bypass
- Temperature Sensor + Hub
- Population Options:
  1)  If using the flash, all switches should be populated.
  2)  If not using the flash, the switch bypass resistors can be populated to 
  maintain cape compatibility.
- I2C Address: 0x48
- TPM
- I2C Address: 0x29
- Switch bypass
- SiP Temp Sensor
- Due to routing constraints, D5+, D6+ and D7+ are not used. | Due to routing constraints, D5+, D6+ and D7+ are not used.
- Suitable alternate parts:
  
  Microchip AT97SC3205T-G3M4C00B
- 10/12 | 11/12 | 12/12
- NOTE: Due to part sourcing issues, both the USB2534 and USB2514B devices are supported.
  See compatibility note below to understand the population requirements to support each device.
- microHDMI connector has 
  slotted thru-holes.
- 4- Port USB Hub | Ethernet | HDMI
- I2C Address: 0x70
- NOTE: Only 500mA is supplied for all 4 ports.
  Therefore, battery charging is disabled
  for all ports.
- NOTE:  All ports are always powered.
- For the TPD4E05 parts, you can route
  through the NC pins.  These pins are next
  to the signal pins and connected to reduce
  DRC errors in layout.
- Ethernet Connector:
    VCC pin is exposed but should be left floating
    for proper connector operation.
- External HDMI audio clock (24.576MHz)
- Configuration
- USB_I2C_SDA
- USB_I2C_SCL
- NOTE:  USB2514B Compatibility
  
  Part     USB2514B    USB2534
  R8       0 ohm            DNP
  C100   0.1 uF            DNP
  C101   1 uF               DNP
  
  R166   100k ohm       50k ohm
  R128   0 ohm            1.5k ohm
  D10     0 ohm            LED
- Configuration
- External HDMI clock (12MHz)
- Ethernet PHY Address: 0x4
    This address must match the PHY address
    defined in the device tree.  If your design
    has more than one Ethernet PHY, the PHY
    address for each PHY must be different.
- PHY_ADDR0
- PHY_ADDR1
- PHY_ADDR2
- MODE[0]
- MODE[1]
- MODE[2]
- MODE[3]
- IO_VOLT_SEL
- 7/12 | 8/12 | 9/12
- SiP GND & Misc | Boot configuration | Cape Headers
- Micro SD card slot
- SYSBOOT[15:0] functionality can be found
  in the "SYSBOOT Configuration Pins" section
  of the AM335x TRM (spruh73)
- SYSBOOT[15:0] = 0x401C (default)
    - Boot Order: MMC1, MMC0, UART0, USB0
  
  SYSBOOT[15:0] = 0x4018 (SD boot)
    - Boot Order: SPI0, MMC0, USB0, UART0
- These connections show which pads were routed through in the layout to reduce DRCs.
- eMMC
- Configuration:
    - 24 MHz Crystal (SYSBOOT[14:15] = 01b)
    - CLKOUT1 disabled (SYSBOOT[5] = 0b)
- JTAG Header
- Half of these resistors, i.e. the ones marked 
  with 'DNI', can be removed.  Only 16 resistors 
  are needed in order to select the default boot 
  mode.  The button above is used to choose an 
  optional SD card boot mode.
- Generic EMMC 5.x Footprint
- Mounting Holes | Fiducials | User LEDs
- While the OSD3358-SM-RED uses 6/6 mil
  trace/space routing rules, we switched to
  5/5mil routing rules for traces within the
  eMMC BGA to accomodate larger 12mil
  BGA landing pads.  For us, this gave greater 
  access to manufacturers and we did not
  want to modify the rest of the design. 
  
  In your design, you can reduce the eMMC
  BGA pads to 9.65mm (see alternate 
  footprint in the library) and use 6/6mil 
  routing rules or you can use 5/5 for the
  entire design.  Please check with your 
  manufacturer for the best set of design rules.
- NOTE 7:  
  
  Do not route through
  RFU / VSF pins.
        
  All other pins are NC and 
  can be routed through.
- Mounting holes and other connector shields are part
  of a ground ring, CGND.  This ring is connected to 
  ground via a resistor on Page 1.
- Only connect EMU2, EMU3 and EMU4 if you plan to use advanced JTAG features 
  (HS-RTDX, Core Trace, System Trace, etc) of higher end debuggers:
  
      - http://processors.wiki.ti.com/index.php/JTAG_Connectors
      - http://processors.wiki.ti.com/index.php/XDS_Target_Connection_Guide
- Suitable alternate parts:
  
  1. WESTERN DIGITAL DEUTSCHLAND SDIN8DE2-16G-XI
  2. SDIN8DE2-16G (Rev3 uses this)
  
  Please choose an appropriate 
  footprint compatible eMMC based on size and availability.
- 4/12 | 5/12 | 6/12
- Power & Reset | Clocks, Analog & USB | SiP Interfaces
- Power input protection.  Adjust 
  according to your application.
- Rev 4:  Load Switch added to mitigate 
  PMIC lockup due to VIN Brownout 
  fault. See Notes on Page 12.
- R168 can be populated with a resistor
  in case the load switch does not have QOD
  or implement your own QOD circuit.
- Octavo Systems OSD335x-SM
  Reference, Evaluation and Development (RED) Platform
  
  (c) Copyright, Octavo Systems LLC, 2017
        All Rights Reserved.
- The values for C7 and C12 can be calculated using
  information in FAQ: https://octavosystems.com/faqs/design-oscillator-circuit-osd335x-family-devices/#more-3862
- Clock resistors R32 and R24 may not be needed in your design.
  See https://octavosystems.com/osd335x/clock/ for more information.
- UART0 debug header
- If the analog interface is not used, 
  then VREFP and VREFN should be 
  shorted to AGND.
- THERE IS NO WARRANTY FOR THIS DESIGN, TO THE EXTENT 
  PERMITTED BY APPLICABLE LAW. EXCEPT WHEN OTHERWISE 
  STATED IN WRITING THE COPYRIGHT HOLDERS AND/OR OTHER 
  PARTIES PROVIDE THE DESIGN *AS IS* WITHOUT WARRANTY OF 
  ANY KIND, EITHER EXPRESSED OR IMPLIED, INCLUDING, BUT NOT 
  LIMITED TO, THE IMPLIED WARRANTIES OF MERCHANTABILITY 
  AND FITNESS A FOR A PARTICULAR PURPOSE. THE ENTIRE RISK 
  AS TO THE QUALITY AND PERFORMANCE OF THE DESIGN IS WITH 
  YOU. SHOULD THE DESIGN PROVE DEFECTIVE, YOU ASSUME THE 
  COST OF ALL NECESSARY SERVICING, REPAIR OR CORRECTION.
- PJ-102BH has 
  slotted thru-holes.
- SYS_ADC_1P8V and AGND_ADC are connected
  to SYS_VDD_1P8V and DGND, respectively, 
  through ferrite beads inside the SiP.  It is 
  not necessary to connect these rails to 
  anything else.  However, bypass capacitors 
  should be added to reduce noise, if needed 
  for your application.
- Rev 4:  PMIC_BAT_SENSE by 
  default shorted to VIN_BAT. For 
  maintain backward compatibility, 
  PMIC_BAT_SENSE can be isolated
  by depopulating the resistor R165.
- Battery Connector
- 32kHz Oscillator is used for the
  RTC.  If your application does 
  not use the RTC, then this 
  can be removed. Please note 
  this may require changes in 
  U-Boot to bypass RTC checks.
- Maximum voltage for the analog 
  inputs is 1.8V.
- DCAN
- The eMMC_RSTN signal no long uses an open-
  drain inverter to control the eMMC reset input
  (See OSD3358 SBC Reference Design).
  This was done to save cost given that there 
  was no software infrastructure in place around
  them eMMC reset.  To put the eMMC in reset
  the pin is now active low.
- 2.4s reset 
  delay @25C
- This is a clamping circuit between the 
  SYS_RTC_1P8V and SYS_VDD3_3P3V outputs of the 
  TPS65217 power management IC inside the 
  OSD335x-SM.  The clamping circuit is related to
  power down issues 
  (see https://octavosystems.com/osd335x/clamping/ 
  for more information). This may not be needed in 
  your application if the power down conditions do 
  not apply to your application.
- Rev 4:  PMIC Reset Supervisor added
  to mitigate PMIC lockup due to VIN
  Brownout fault. See Notes on Page 12.
- AIN7 currently monitors the PMIC voltages 
  via the internal PMIC mux.  See the `Analog 
  Multiplexer' section of the TPS65217 
  datasheet.  For the internal PMIC voltages, 
  there are dividers within the PMIC to keep 
  the montiored voltages under 1.8V.  However, 
  PMIC_MUX_IN does not have any dividers 
  and must be less than 1.8V.  By default, 
  PMIC_MUX_OUT is Hi-Z.  The MUXCTRL 
  register in the PMIC is used to select the 
  PMIC_MUX_OUT voltage path.
- USBx_VBUS is a voltage sense input. It is
  NOT a power output pin. The USBx peripheral
  will be enabled only if a valid voltage
  ( >=4.4V ) is present on this pin. For more
  info see "USB Circuitry" article on 
  www.octavosystems.com/app_notes
- Rev 4:  Reset Supervisor U4 repurposed 
  to monitor VIN_AC to prevent PMIC 
  lockup due to VIN Brownout fault.  
  Reset supervisor from previous
  revisions can still be used if desired.
- SYS_VDD1_3P3V is a 3.3V output of the 
  OSD3358-512M-BSM.  A divide by 2 resistor 
  divider is used to ensure that the PMIC_MUX_IN 
  voltage does not exceed 1.8V.  It is not 
  necessary to monitor the TL5209 LDO output 
  and this can be removed if desired.
- The 0 Ohm resistor (R10) on the 
  VBUS input can be replaced with 
  a ferrite bead for noise 
  suppresion or a solder bridge 
  for cost reduction.
- The OSD335x-SM contains 4.7k 
  pull-up resistors on I2C0. 
  External resistors added so 
  that pull-up strength can be 
  changed due to layout or 
  other requirements.
- I2C0 Devices inside SiP:
- TPS65217 I2C Address: 0x24
- EEPROM I2C Address: 0x50
- Per the TPD4S012 datasheet, D-, D+ 
  and ID have the same ESD circuitry.
  Therefore, to ease routing, D- and D+
  have been swapped from the default
  mapping.
- Reset inputs:
      1) Manual push-button
      2) PMIC_PGOOD
- Resistor and capacitor footprints 
  are added to CLKOUT1/CLKOUT2 in 
  case EMI suppression is needed.
- RTC_KALDO_ENN is grounded thru a 10K ohm resistor so that 
  the internal RTC LDO is enabled and CAP_VDD_RTC does not 
  need to be connected to VDD_CORE.
- USB Client
- Nets like CLKOUT2, GPIO0_7 and GPIO1_16 are resistor muxed to increase the
  functionality of the Cape Headers.  This is not needed if your application 
  does not require Cape Header compatibility.
- To Print:  Use 8.5"x11" paper in landscape; 0.69 scaling factor.
- 1/12 | 2/12 | 3/12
